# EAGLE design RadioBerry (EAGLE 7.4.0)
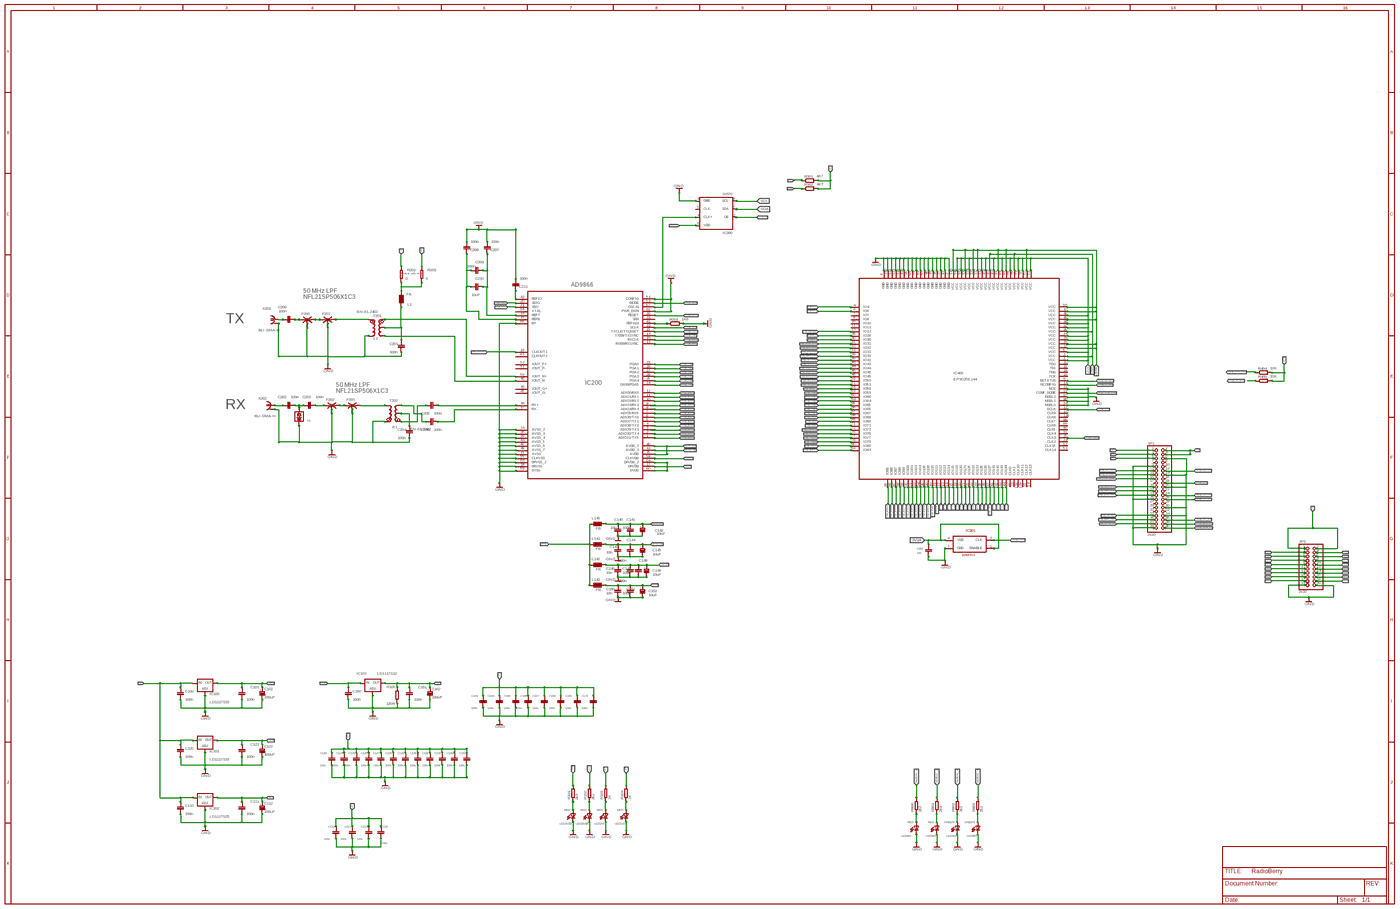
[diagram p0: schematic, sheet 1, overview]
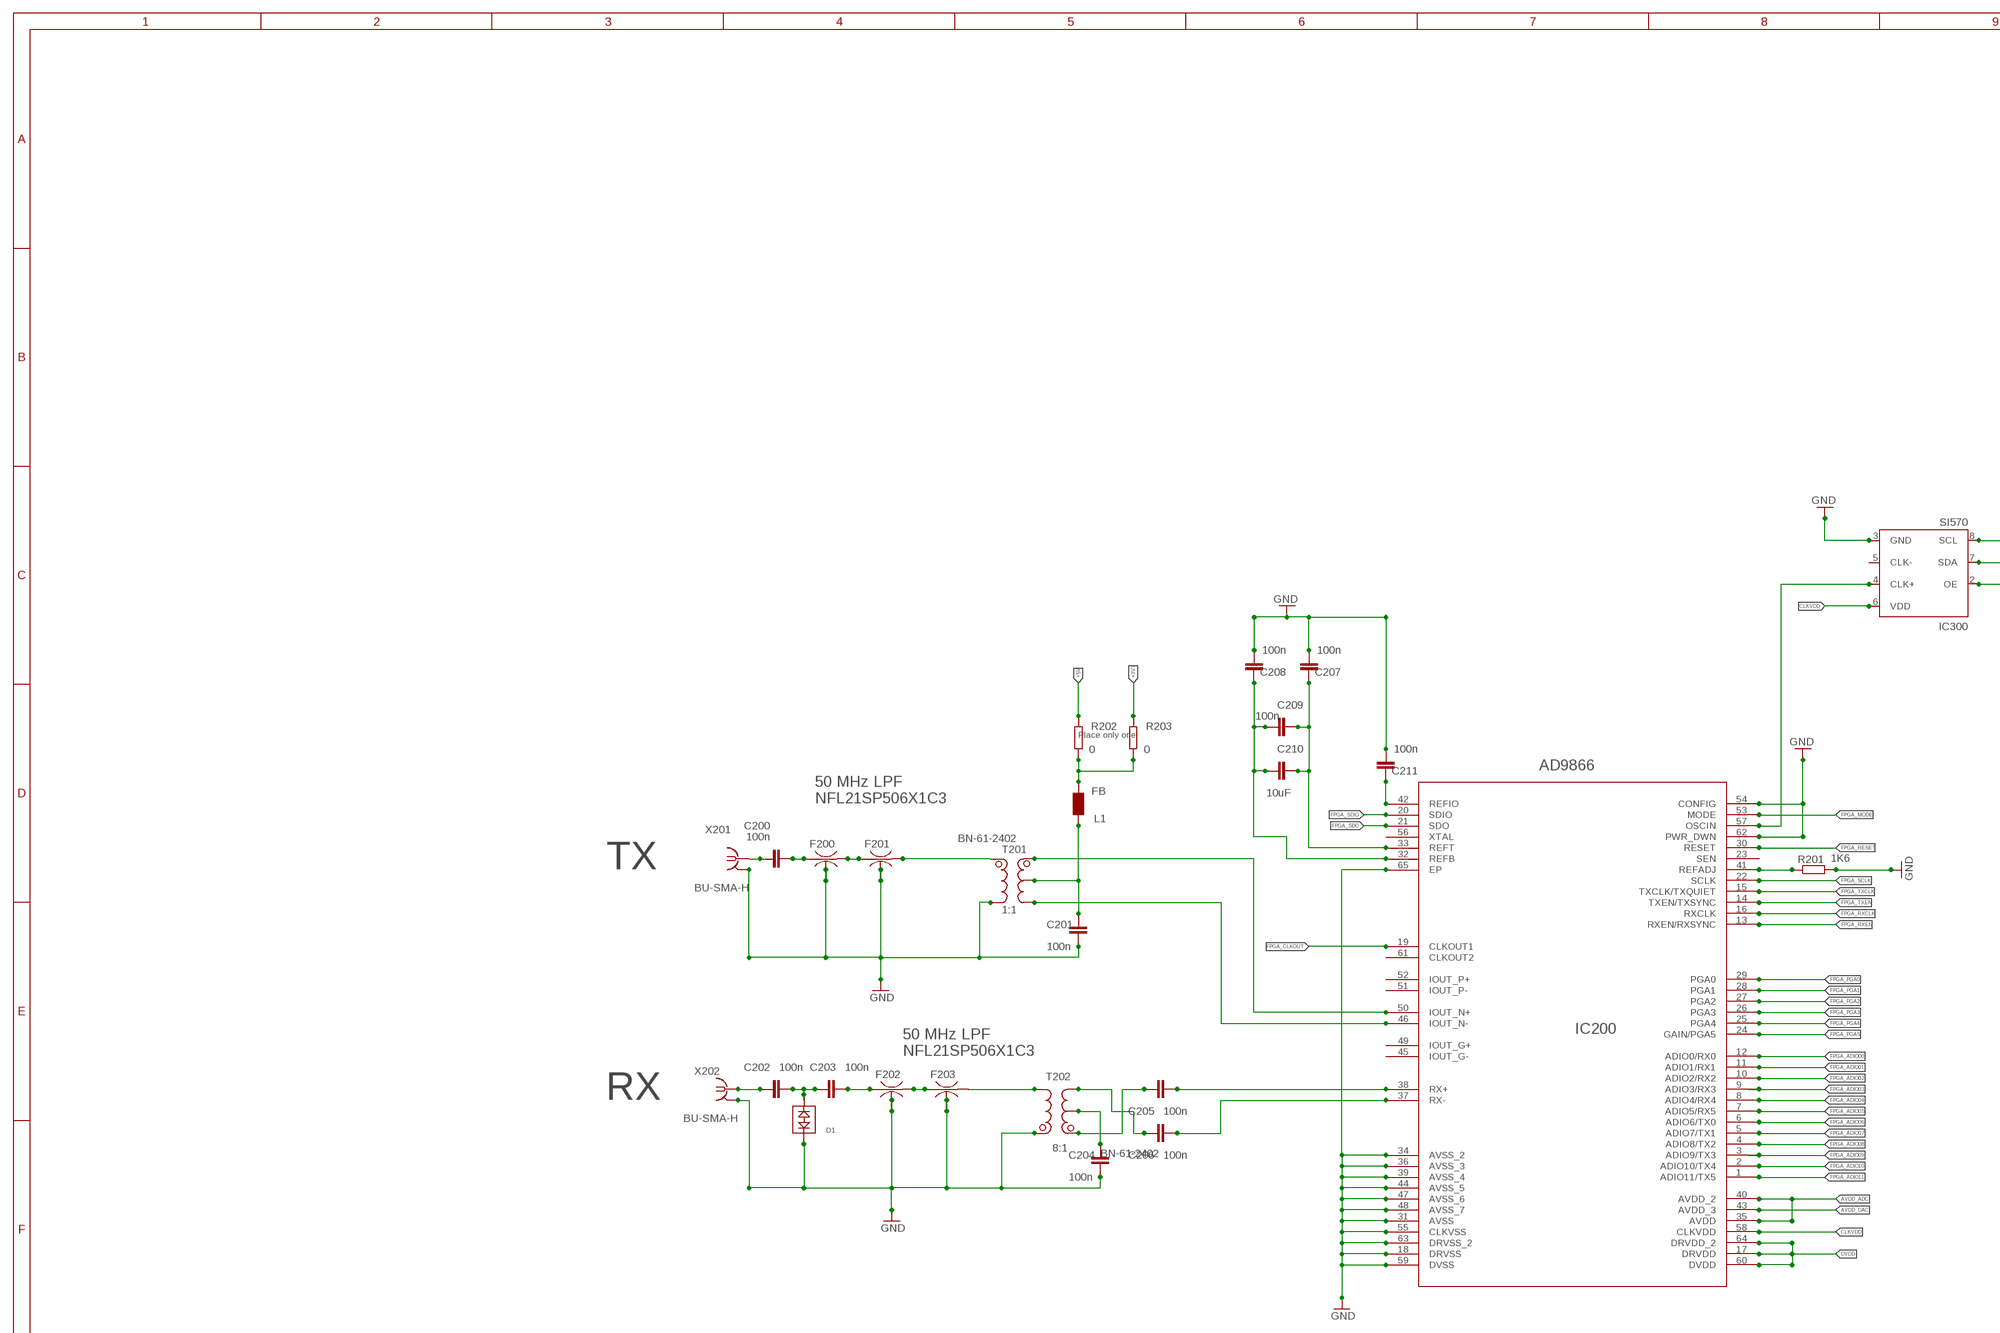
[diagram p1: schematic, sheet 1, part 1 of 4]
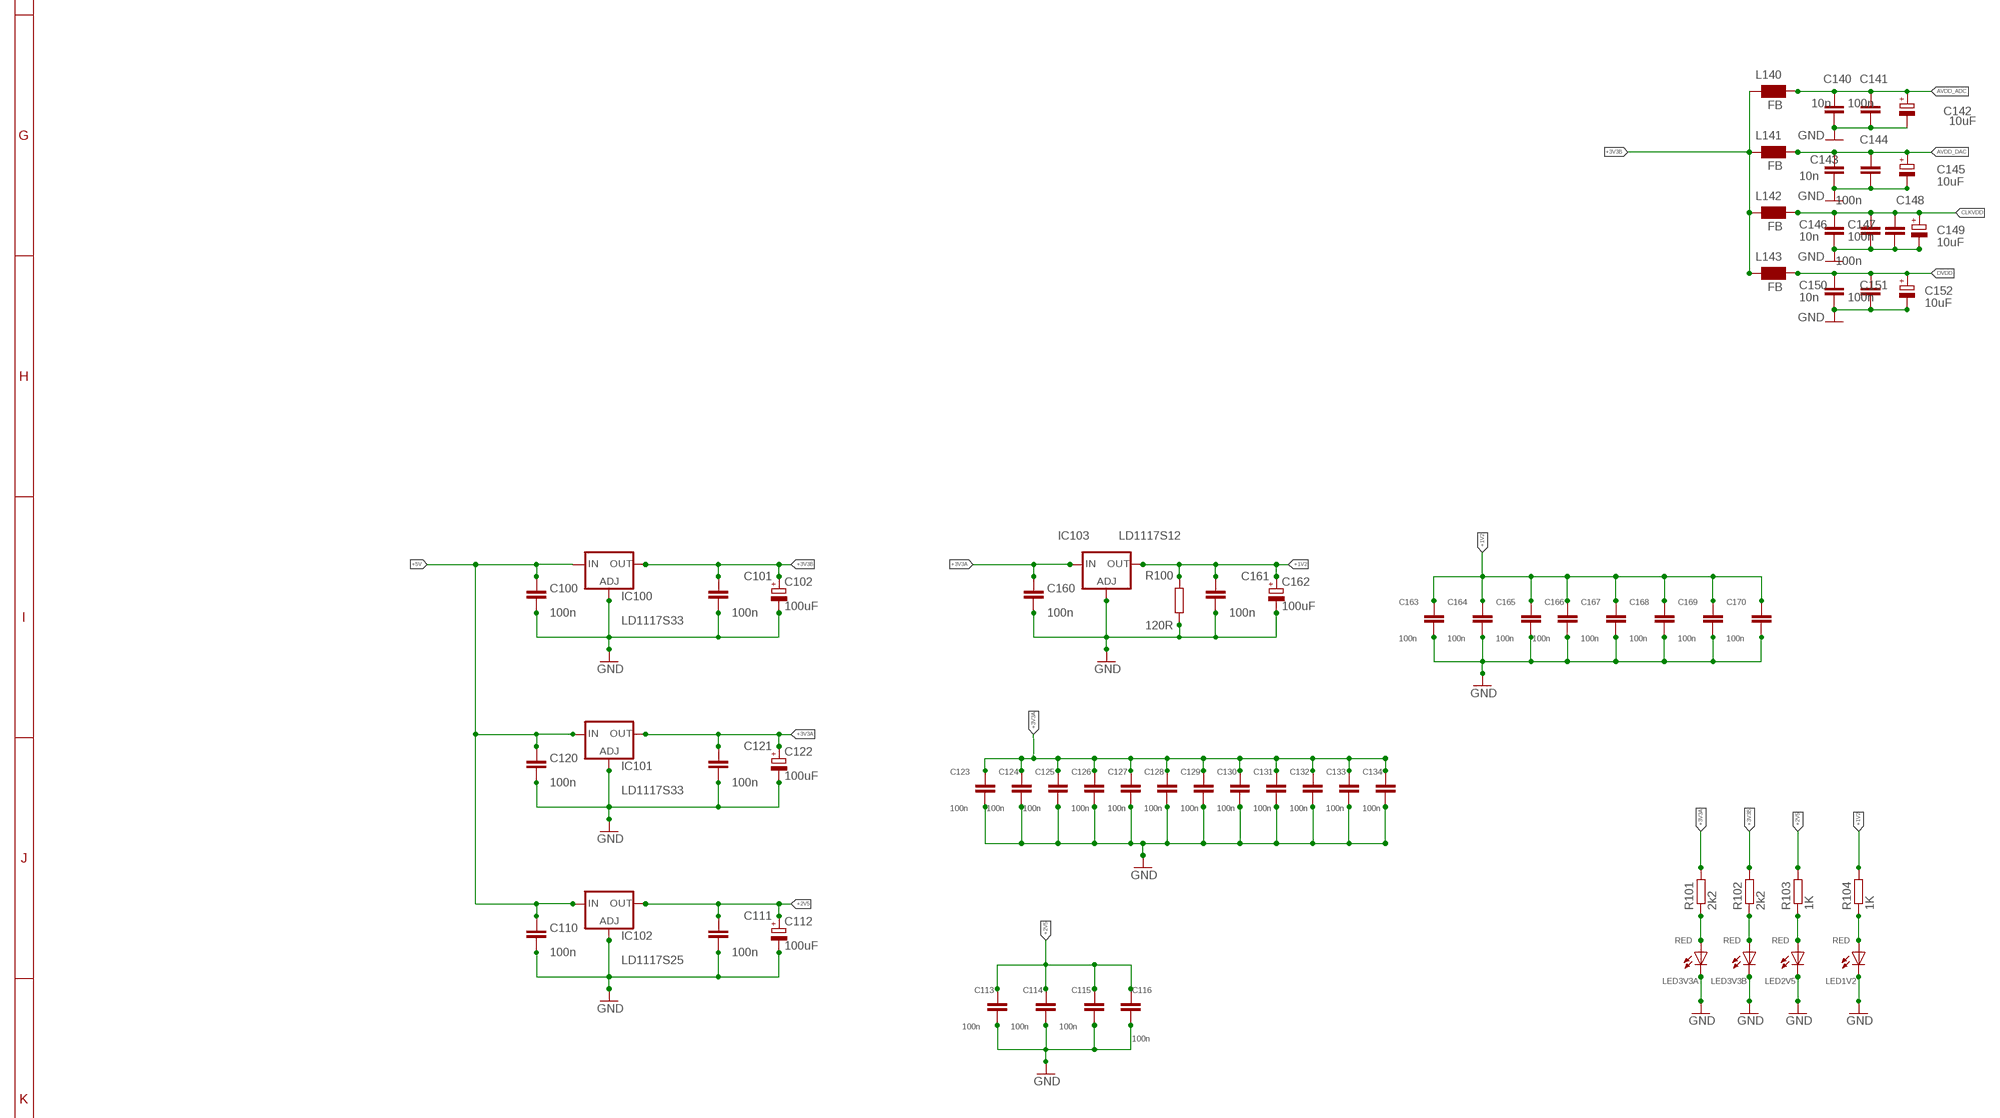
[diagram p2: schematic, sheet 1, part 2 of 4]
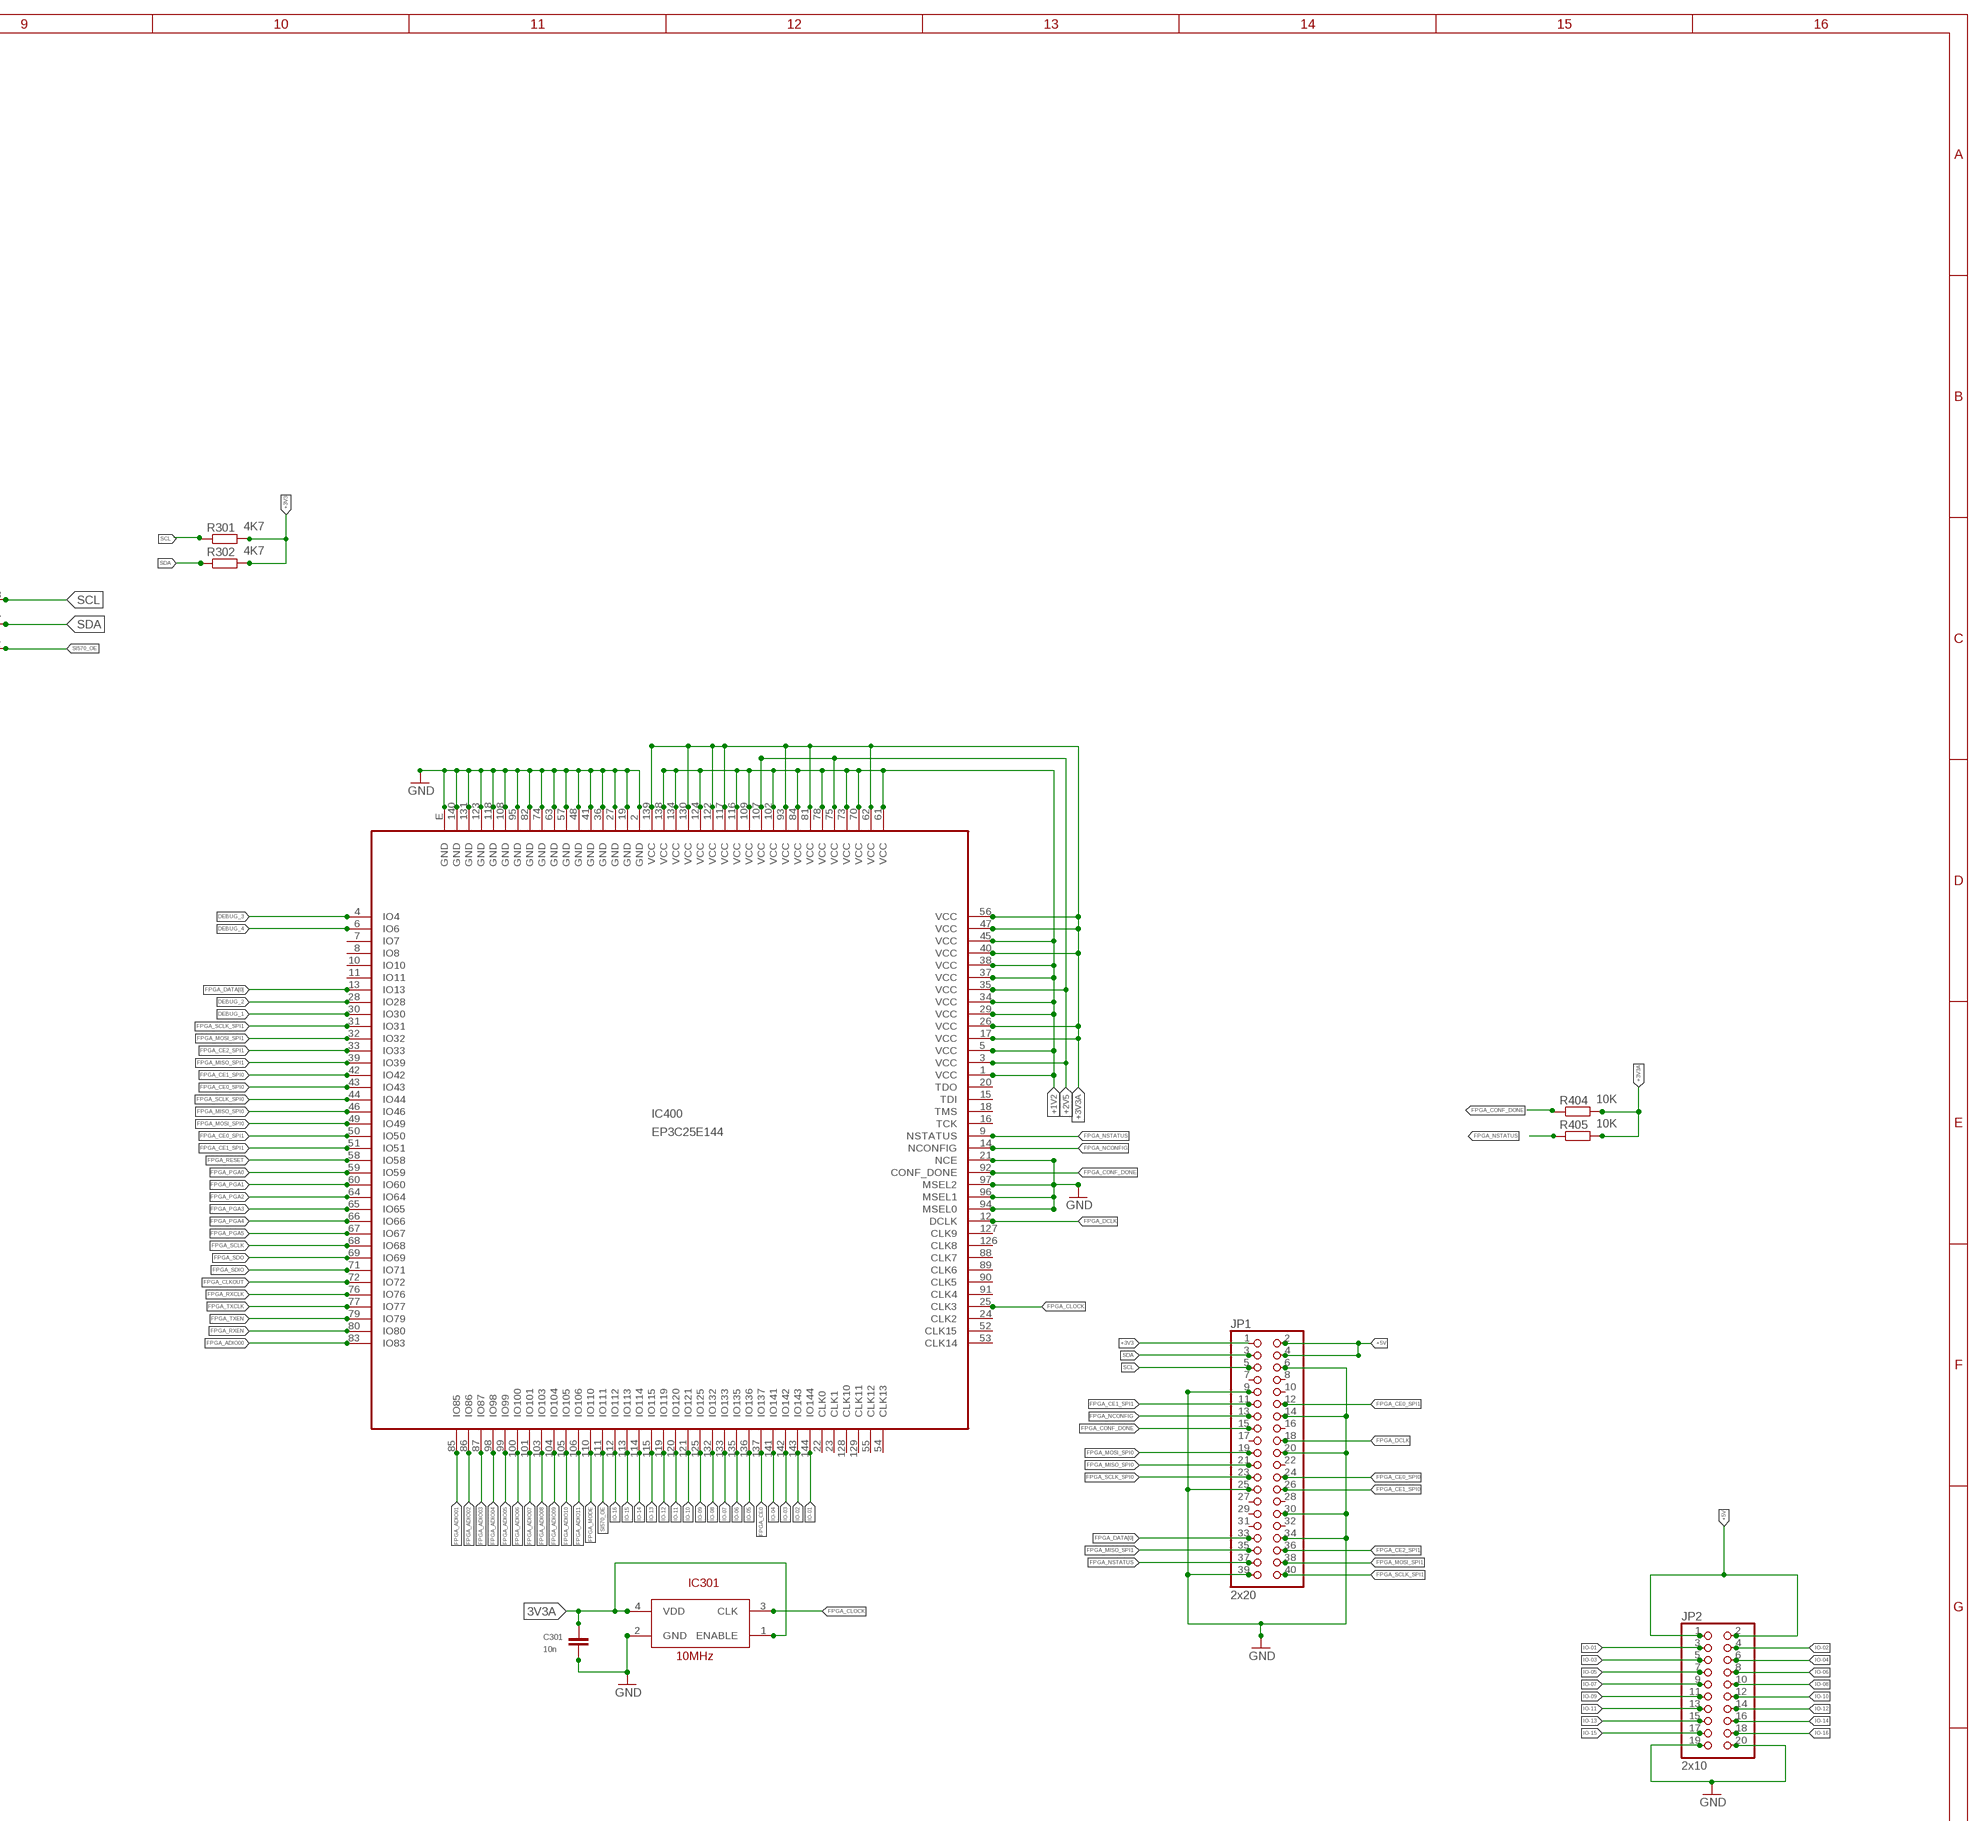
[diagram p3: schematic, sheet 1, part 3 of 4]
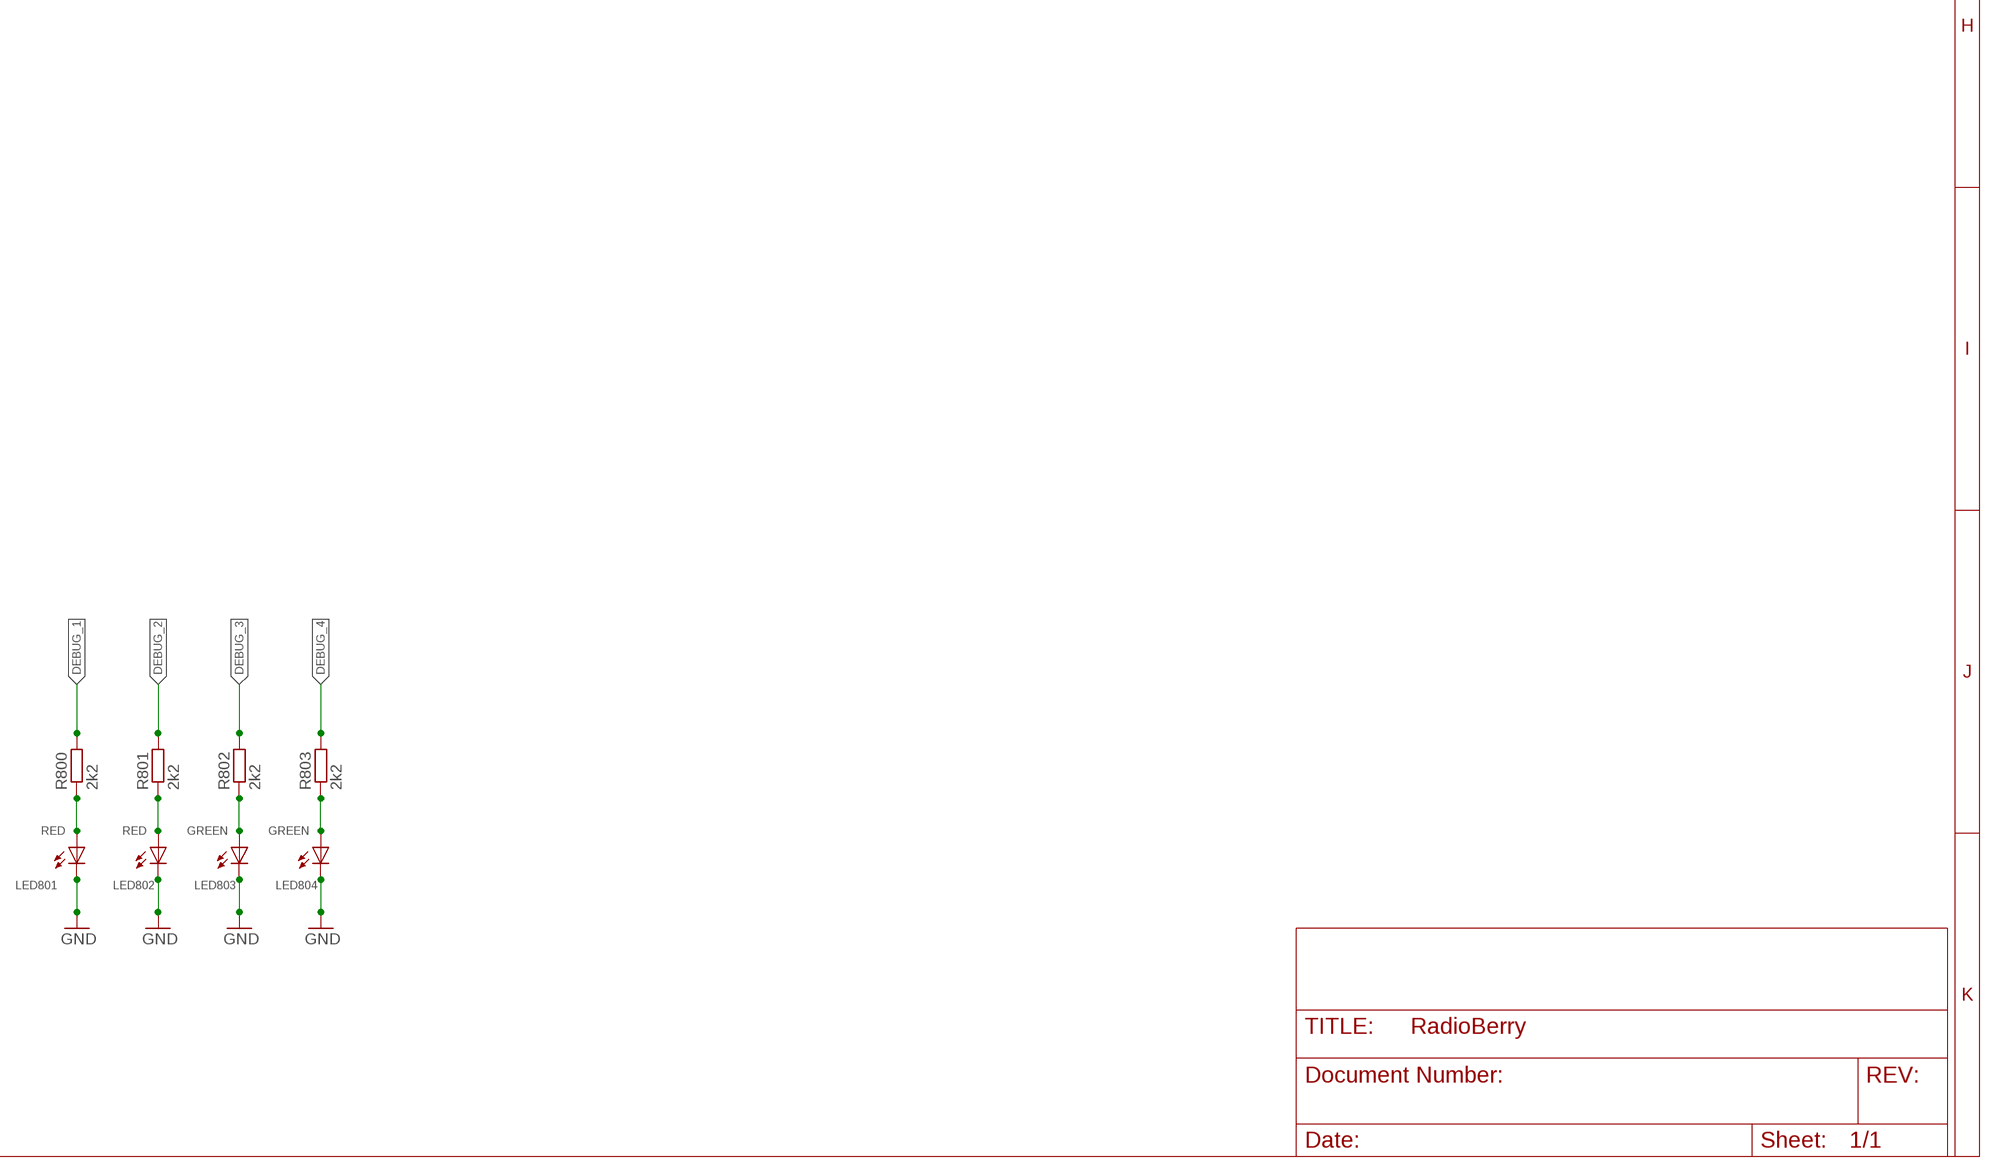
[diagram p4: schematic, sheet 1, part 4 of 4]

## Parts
C100  100n  C-EUC0603  [C0603]
C101  100n  C-EUC0603  [C0603]
C102  100uF  CPOL-EUSMCA  [SMC_A]
C110  100n  C-EUC0603  [C0603]
C111  100n  C-EUC0603  [C0603]
C112  100uF  CPOL-EUSMCA  [SMC_A]
C113  100n  C-EUC0603  [C0603]
C114  100n  C-EUC0603  [C0603]
C115  100n  C-EUC0603  [C0603]
C116  100n  C-EUC0603  [C0603]
C120  100n  C-EUC0603  [C0603]
C121  100n  C-EUC0603  [C0603]
C122  100uF  CPOL-EUSMCA  [SMC_A]
C123  100n  C-EUC0603  [C0603]
C124  100n  C-EUC0603  [C0603]
C125  100n  C-EUC0603  [C0603]
C126  100n  C-EUC0603  [C0603]
C127  100n  C-EUC0603  [C0603]
C128  100n  C-EUC0603  [C0603]
C129  100n  C-EUC0603  [C0603]
C130  100n  C-EUC0603  [C0603]
C131  100n  C-EUC0603  [C0603]
C132  100n  C-EUC0603  [C0603]
C133  100n  C-EUC0603  [C0603]
C134  100n  C-EUC0603  [C0603]
C140  10n  C-EUC0603  [C0603]
C141  100n  C-EUC0603  [C0603]
C142  10uF  CPOL-EUSMCA  [SMC_A]
C143  10n  C-EUC0603  [C0603]
C144  100n  C-EUC0603  [C0603]
C145  10uF  CPOL-EUSMCA  [SMC_A]
C146  10n  C-EUC0603  [C0603]
C147  100n  C-EUC0603  [C0603]
C148  100n  C-EUC0603  [C0603]
C149  10uF  CPOL-EUSMCA  [SMC_A]
C150  10n  C-EUC0603  [C0603]
C151  100n  C-EUC0603  [C0603]
C152  10uF  CPOL-EUSMCA  [SMC_A]
C160  100n  C-EUC0603  [C0603]
C161  100n  C-EUC0603  [C0603]
C162  100uF  CPOL-EUSMCA  [SMC_A]
C163  100n  C-EUC0603  [C0603]
C164  100n  C-EUC0603  [C0603]
C165  100n  C-EUC0603  [C0603]
C166  100n  C-EUC0603  [C0603]
C167  100n  C-EUC0603  [C0603]
C168  100n  C-EUC0603  [C0603]
C169  100n  C-EUC0603  [C0603]
C170  100n  C-EUC0603  [C0603]
C200  100n  C-EUC0603  [C0603]
C201  100n  C-EUC0603  [C0603]
C202  100n  C-EUC0603  [C0603]
C203  100n  C-EUC0603  [C0603]
C204  100n  C-EUC0603  [C0603]
C205  100n  C-EUC0603  [C0603]
C206  100n  C-EUC0603  [C0603]
C207  100n  C-EUC0603  [C0603]
C208  100n  C-EUC0603  [C0603]
C209  100n  C-EUC0603  [C0603]
C210  10uF  C-EUC1206  [C1206]
C211  100n  C-EUC0603  [C0603]
C301  10n  C-EUC0603  [C0603]
D1  GBLC03C  [SOD-323]
F200  NFM21C  [NFM21C]
F201  NFM21C  [NFM21C]
F202  NFM21C  [NFM21C]
F203  NFM21C  [NFM21C]
IC100  LD1117S33  LD117AS33TR  [SOT223]
IC101  LD1117S33  LD117AS33TR  [SOT223]
IC102  LD1117S25  LD117AS33TR  [SOT223]
IC103  LD1117S12  LD117AS12TR  [SOT223]
IC200  AD9866  [CP_64_3]
IC300  SI570  [8-PIN]
IC301  10MHz  CLOCK  [MODEL625]
IC400  EP3C25E144  [EQFP144]
JP1  2x20  PINHD-2X20  [2X20]
JP2  2x10  PINHD-2X10  [2X10]
L1  FB  WE-CBF_0805  [0805]
L140  FB  WE-CBF_0805  [0805]
L141  FB  WE-CBF_0805  [0805]
L142  FB  WE-CBF_0805  [0805]
L143  FB  WE-CBF_0805  [0805]
LED1V2  RED  LEDCHIP-LED0805  [CHIP-LED0805]
LED2V5  RED  LEDCHIP-LED0805  [CHIP-LED0805]
LED3V3A  RED  LEDCHIP-LED0805  [CHIP-LED0805]
LED3V3B  RED  LEDCHIP-LED0805  [CHIP-LED0805]
LED801  RED  LEDCHIP-LED0805  [CHIP-LED0805]
LED802  RED  LEDCHIP-LED0805  [CHIP-LED0805]
LED803  GREEN  LEDCHIP-LED0805  [CHIP-LED0805]
LED804  GREEN  LEDCHIP-LED0805  [CHIP-LED0805]
R100  120R  R-EU_R0805  [R0805]
R101  2k2  R-EU_R0805  [R0805]
R102  2k2  R-EU_R0805  [R0805]
R103  1K  R-EU_R0805  [R0805]
R104  1K  R-EU_R0805  [R0805]
R201  1K6  R-EU_R0805  [R0805]
R202  0  R-EU_R0805  [R0805]
R203  0  R-EU_R0805  [R0805]
R301  4K7  R-EU_R0805  [R0805]
R302  4K7  R-EU_R0805  [R0805]
R404  10K  R-EU_R0805  [R0805]
R405  10K  R-EU_R0805  [R0805]
R800  2k2  R-EU_R0805  [R0805]
R801  2k2  R-EU_R0805  [R0805]
R802  2k2  R-EU_R0805  [R0805]
R803  2k2  R-EU_R0805  [R0805]
T201  BN-61-2402  T1-1TDIL  [DIL06]
T202  BN-61-2402  T1-1TDIL  [DIL06]
X201  BU-SMA-H  [BU-SMA-H]
X202  BU-SMA-H  [BU-SMA-H]

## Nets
3V3A: C301.2 IC301.1(ENABLE) IC301.4(VDD)
+1V2: C161.2 C162.+ C163.2 C164.2 C165.2 C166.2 C167.2 C168.2 C169.2 C170.2 IC103.4(OUT) IC400.1(VCC) IC400.5(VCC) IC400.29(VCC) IC400.34(VCC) IC400.37(VCC) IC400.38(VCC) IC400.45(VCC) IC400.61(VCC) IC400.70(VCC) IC400.73(VCC) IC400.78(VCC) IC400.84(VCC) IC400.102(VCC) IC400.109(VCC) IC400.116(VCC) IC400.124(VCC) IC400.134(VCC) IC400.138(VCC) R100.2 R104.2
+2V5: C111.2 C112.+ C113.2 C114.2 C115.2 C116.2 IC102.4(OUT) IC400.3(VCC) IC400.35(VCC) IC400.75(VCC) IC400.107(VCC) R103.2
+3V3: JP1.1 R203.2 R301.2 R302.2
+3V3A: C121.2 C122.+ C123.2 C124.2 C125.2 C126.2 C127.2 C128.2 C129.2 C130.2 C131.2 C132.2 C133.2 C134.2 C160.2 IC101.4(OUT) IC103.3(IN) IC400.17(VCC) IC400.26(VCC) IC400.40(VCC) IC400.47(VCC) IC400.56(VCC) IC400.62(VCC) IC400.81(VCC) IC400.93(VCC) IC400.117(VCC) IC400.122(VCC) IC400.130(VCC) IC400.139(VCC) R101.2 R404.2 R405.2
+3V3B: C101.2 C102.+ IC100.4(OUT) L140.1 L141.1 L142.1 L143.1 R102.2
+5V: C100.2 C110.2 C120.2 IC100.3(IN) IC101.3(IN) IC102.3(IN) JP1.2 JP1.4 JP2.1 JP2.2 R202.2
AVDD_ADC: C140.2 C141.2 C142.+ IC200.35(AVDD) IC200.40(AVDD_2) L140.2
AVDD_DAC: C143.2 C144.2 C145.+ IC200.43(AVDD_3) L141.2
CLK: IC200.57(OSCIN) IC300.4(CLK+)
CLKVDD: C146.2 C147.2 C148.2 C149.+ IC200.58(CLKVDD) IC300.6(VDD) L142.2
DEBUG_1: IC400.30(IO30) R800.2
DEBUG_2: IC400.28(IO28) R801.2
DEBUG_3: IC400.4(IO4) R802.2
DEBUG_4: IC400.6(IO6) R803.2
DVDD: C150.2 C151.2 C152.+ IC200.17(DRVDD) IC200.60(DVDD) IC200.64(DRVDD_2) L143.2
FPGA_ADIO00: IC200.12(ADIO0/RX0) IC400.83(IO83)
FPGA_ADIO01: IC200.11(ADIO1/RX1) IC400.85(IO85)
FPGA_ADIO02: IC200.10(ADIO2/RX2) IC400.86(IO86)
FPGA_ADIO03: IC200.9(ADIO3/RX3) IC400.87(IO87)
FPGA_ADIO04: IC200.8(ADIO4/RX4) IC400.98(IO98)
FPGA_ADIO05: IC200.7(ADIO5/RX5) IC400.99(IO99)
FPGA_ADIO06: IC200.6(ADIO6/TX0) IC400.100(IO100)
FPGA_ADIO07: IC200.5(ADIO7/TX1) IC400.101(IO101)
FPGA_ADIO08: IC200.4(ADIO8/TX2) IC400.103(IO103)
FPGA_ADIO09: IC200.3(ADIO9/TX3) IC400.104(IO104)
FPGA_ADIO10: IC200.2(ADIO10/TX4) IC400.105(IO105)
FPGA_ADIO11: IC200.1(ADIO11/TX5) IC400.106(IO106)
FPGA_CE0: IC400.137(IO137)
FPGA_CE0_SPI0: IC400.43(IO43) JP1.24
FPGA_CE0_SPI1: IC400.50(IO50) JP1.12
FPGA_CE1_SPI0: IC400.42(IO42) JP1.26
FPGA_CE1_SPI1: IC400.51(IO51) JP1.11
FPGA_CE2_SPI1: IC400.33(IO33) JP1.36
FPGA_CLKOUT: IC200.19(CLKOUT1) IC400.72(IO72)
FPGA_CLOCK: IC301.3(CLK) IC400.25(CLK3)
FPGA_CONF_DONE: IC400.92(CONF_DONE) JP1.15 R404.1
FPGA_DATA[0]: IC400.13(IO13) JP1.33
FPGA_DCLK: IC400.12(DCLK) JP1.18
FPGA_MISO_SPI0: IC400.46(IO46) JP1.21
FPGA_MISO_SPI1: IC400.39(IO39) JP1.35
FPGA_MODE: IC200.53(MODE) IC400.110(IO110)
FPGA_MOSI_SPI0: IC400.49(IO49) JP1.19
FPGA_MOSI_SPI1: IC400.32(IO32) JP1.38
FPGA_NCONFIG: IC400.14(NCONFIG) JP1.13
FPGA_NSTATUS: IC400.9(NSTATUS) JP1.37 R405.1
FPGA_PGA0: IC200.29(PGA0) IC400.59(IO59)
FPGA_PGA1: IC200.28(PGA1) IC400.60(IO60)
FPGA_PGA2: IC200.27(PGA2) IC400.64(IO64)
FPGA_PGA3: IC200.26(PGA3) IC400.65(IO65)
FPGA_PGA4: IC200.25(PGA4) IC400.66(IO66)
FPGA_PGA5: IC200.24(GAIN/PGA5) IC400.67(IO67)
FPGA_RESET: IC200.30(RESET) IC400.58(IO58)
FPGA_RXCLK: IC200.16(RXCLK) IC400.76(IO76)
FPGA_RXEN: IC200.13(RXEN/RXSYNC) IC400.80(IO80)
FPGA_SCLK: IC200.22(SCLK) IC400.68(IO68)
FPGA_SCLK_SPI0: IC400.44(IO44) JP1.23
FPGA_SCLK_SPI1: IC400.31(IO31) JP1.40
FPGA_SDIO: IC200.20(SDIO) IC400.71(IO71)
FPGA_SDO: IC200.21(SDO) IC400.69(IO69)
FPGA_TXCLK: IC200.15(TXCLK/TXQUIET) IC400.77(IO77)
FPGA_TXEN: IC200.14(TXEN/TXSYNC) IC400.79(IO79)
GND: C100.1 C101.1 C102.- C110.1 C111.1 C112.- C113.1 C114.1 C115.1 C116.1 C120.1 C121.1 C122.- C123.1 C124.1 C125.1 C126.1 C127.1 C128.1 C129.1 C130.1 C131.1 C132.1 C133.1 C134.1 C140.1 C141.1 C142.- C143.1 C144.1 C145.- C146.1 C147.1 C148.1 C149.- C150.1 C151.1 C152.- C160.1 C161.1 C162.- C163.1 C164.1 C165.1 C166.1 C167.1 C168.1 C169.1 C170.1 C201.1 C204.1 C207.1 C208.1 C211.1 C301.1 D1.B F200.2@1 F200.2@2 F201.2@1 F201.2@2 F202.2@1 F202.2@2 F203.2@1 F203.2@2 IC100.1(ADJ) IC101.1(ADJ) IC102.1(ADJ) IC103.1(ADJ) IC200.18(DRVSS) IC200.31(AVSS) IC200.34(AVSS_2) IC200.36(AVSS_3) IC200.39(AVSS_4) IC200.44(AVSS_5) IC200.47(AVSS_6) IC200.48(AVSS_7) IC200.54(CONFIG) IC200.55(CLKVSS) IC200.59(DVSS) IC200.62(PWR_DWN) IC200.63(DRVSS_2) IC200.65(EP) IC300.3(GND) IC301.2(GND) IC400.2(GND) IC400.19(GND) IC400.21(NCE) IC400.27(GND) IC400.36(GND) IC400.41(GND) IC400.48(GND) IC400.57(GND) IC400.63(GND) IC400.74(GND) IC400.82(GND) IC400.94(MSEL0) IC400.95(GND) IC400.96(MSEL1) IC400.97(MSEL2) IC400.108(GND) IC400.118(GND) IC400.123(GND) IC400.131(GND) IC400.140(GND) IC400.E(GND) JP1.6 JP1.9 JP1.14 JP1.20 JP1.25 JP1.30 JP1.34 JP1.39 JP2.19 JP2.20 LED1V2.C LED2V5.C LED3V3A.C LED3V3B.C LED801.C LED802.C LED803.C LED804.C R100.1 R201.2 T201.1(P2) T202.3(P1) X201.2 X201.3 X201.4 X201.5 X202.2 X202.3 X202.4 X202.5
IO-01: IC400.144(IO144) JP2.3
IO-02: IC400.143(IO143) JP2.4
IO-03: IC400.142(IO142) JP2.5
IO-04: IC400.141(IO141) JP2.6
IO-05: IC400.136(IO136) JP2.7
IO-06: IC400.135(IO135) JP2.8
IO-07: IC400.133(IO133) JP2.9
IO-08: IC400.132(IO132) JP2.10
IO-09: IC400.125(IO125) JP2.11
IO-10: IC400.121(IO121) JP2.12
IO-11: IC400.120(IO120) JP2.13
IO-12: IC400.119(IO119) JP2.14
IO-13: IC400.115(IO115) JP2.15
IO-14: IC400.114(IO114) JP2.16
IO-15: IC400.113(IO113) JP2.17
IO-16: IC400.112(IO112) JP2.18
N$1: L1.2 R202.1 R203.1
N$2: F203.3 T202.1(P2)
N$3: C205.2 T202.4(S1)
N$4: C201.2 L1.1 T201.5(ST)
N$5: C202.1 C203.2 D1.A
N$6: IC200.50(IOUT_N+) T201.4(S1)
N$7: IC200.46(IOUT_N-) T201.6(S2)
N$8: C206.2 T202.6(S2)
N$10: LED3V3B.A R102.1
N$11: LED2V5.A R103.1
N$13: C206.1 IC200.37(RX-)
N$14: C204.2 T202.5(ST)
N$15: C205.1 IC200.38(RX+)
N$16: LED801.A R800.1
N$17: LED802.A R801.1
N$18: LED803.A R802.1
N$19: LED804.A R803.1
N$20: LED3V3A.A R101.1
N$23: LED1V2.A R104.1
N$25: F202.3 F203.1
N$28: C202.2 X202.1
N$29: C203.1 F202.1
N$30: C207.2 C209.2 C210.2 IC200.33(REFT)
N$32: C208.2 C209.1 C210.1 IC200.32(REFB)
N$33: C211.2 IC200.42(REFIO)
N$34: IC200.41(REFADJ) R201.1
N$69: C200.2 X201.1
N$71: C200.1 F200.1
N$72: F200.3 F201.1
N$73: F201.3 T201.3(P1)
SCL: IC300.8(SCL) JP1.5 R301.1
SDA: IC300.7(SDA) JP1.3 R302.1
SI570_OE: IC300.2(OE) IC400.111(IO111)
Unconnected: IC200.23(SEN) IC200.45(IOUT_G-) IC200.49(IOUT_G+) IC200.51(IOUT_P-) IC200.52(IOUT_P+) IC200.56(XTAL) IC200.61(CLKOUT2) IC300.5(CLK-) IC400.7(IO7) IC400.8(IO8) IC400.10(IO10) IC400.11(IO11) IC400.15(TDI) IC400.16(TCK) IC400.18(TMS) IC400.20(TDO) IC400.22(CLK0) IC400.23(CLK1) IC400.24(CLK2) IC400.52(CLK15) IC400.53(CLK14) IC400.54(CLK13) IC400.55(CLK12) IC400.88(CLK7) IC400.89(CLK6) IC400.90(CLK5) IC400.91(CLK4) IC400.126(CLK8) IC400.127(CLK9) IC400.128(CLK10) IC400.129(CLK11) JP1.7 JP1.8 JP1.10 JP1.16 JP1.17 JP1.22 JP1.27 JP1.28 JP1.29 JP1.31 JP1.32

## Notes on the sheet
- Configuration
- Place only one
- 50 MHz LPF
  NFL21SP506X1C3
- TX
- 1:1
- 50 MHz LPF
  NFL21SP506X1C3
- RX
- 8:1
- Power Supply
- [100]

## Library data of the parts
C100 C101 C110 C111 C113-C116 C120 C121 C123-C134 C140 C141 C143 C144 C146-C148 C150 C151 C160 C161 C163-C170 C200-C211 C301 = rcl:C-EU: CAPACITOR, European symbol
C102 C112 C122 C142 C145 C149 C152 C162 = rcl:CPOL-EU: POLARIZED CAPACITOR, European symbol
D1 = pa3gsb:GBLC03C
F200-F203 = murata-filter:NFM: EMIFIL(R) (Capacitor type) Single Circuit Type for Signal Lines Source: http://search.murata.co.jp/Ceramy/image/img/PDF/ENG/L0111S0109NFM3DC.pdf
IC100-IC103 = v-reg:LD117A?*: Low drop fixed and adjustable positive voltage regulators 1 A Source: http://www.st.com/stonline/products/literature/ds/7194/ld1117axx.pdf
IC200 = AD9866:AD9866
IC300 = silabs:SI570: ANY-RATE I2C PROGRAMMABLE XO/VCXO Source: si570.pdf; OC_FARNELL: unknown; OC_NEWARK: unknown
IC301 = AVS-Clock:CLOCK
IC400 = altera-cyclone-III:EP3C25E144: EP3C25E144 edit this description Auto generated by make-symbol-device-package-bsdl.ulp Rev. 20 Source: EP3C25E144.bsd http://www.altera.com/support/devices/bsdl/cyclone3/cyc3-index.jsp; MPN: EP3C25E144C8N; OC_FARNELL: 1453474; OC_NEWARK: 51R0605
JP1 = pinhead:PINHD-2X20: PIN HEADER
JP2 = pinhead:PINHD-2X10: PIN HEADER
L1 L140-L143 = wuerth-elektronik:WE-CBF: SMD EMI Suppression Ferrite Beads
LED1V2 LED2V5 LED3V3A LED3V3B LED801-LED804 = led:LED: LED
R100-R104 R201-R203 R301 R302 R404 R405 R800-R803 = rcl:R-EU_: RESISTOR, European symbol
T201 T202 = pa3gsb:T1-1T
X201 X202 = con-coax:BU-SMA-H: FEMALE SMA CONNECTOR; OC_FARNELL: unknown; OC_NEWARK: unknown

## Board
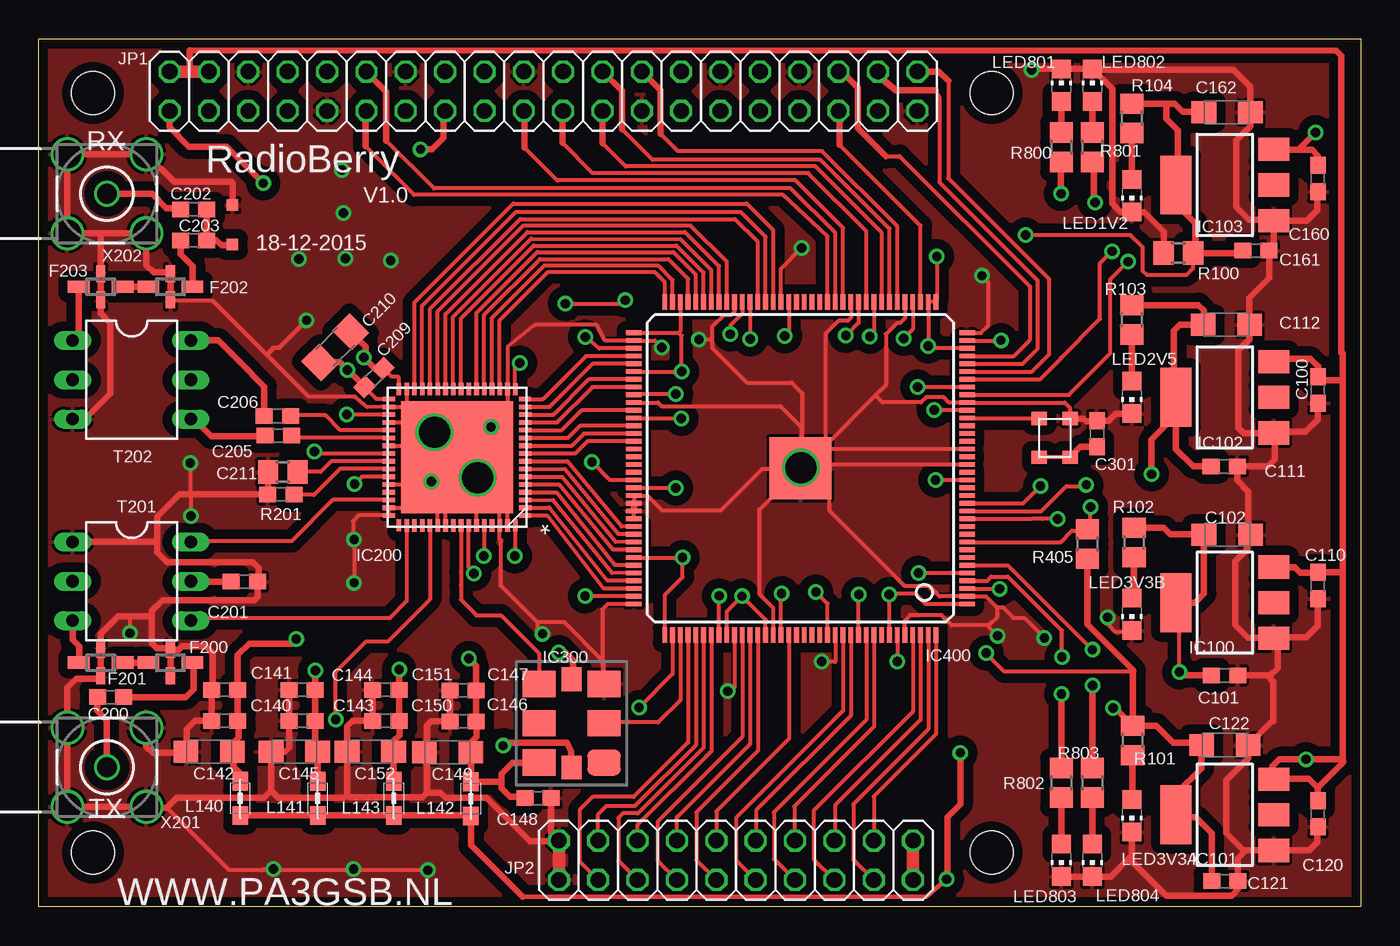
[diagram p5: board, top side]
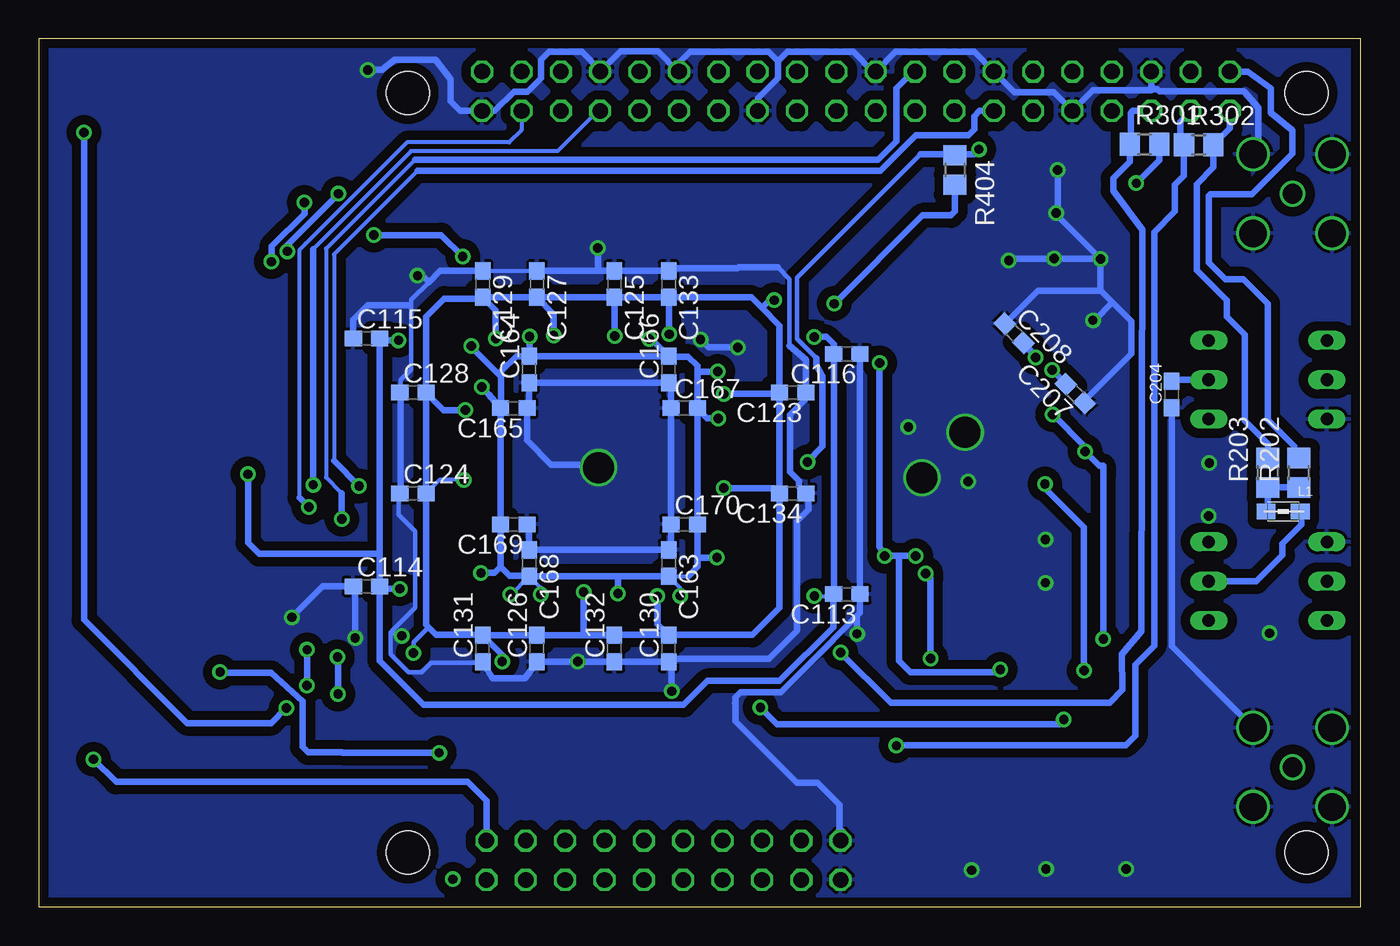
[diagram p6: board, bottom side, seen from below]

Size 85.32 x 56 mm. Coordinates in mm from the lower left corner, seen from the top.
Outline: 0,56 85.32,56 85.32,0 0,0 0,56
Copper layers (1*16): Top 0.018mm / dielectric 1.55mm / Bottom 0.018mm
Design rules "eC-PCB_proto-2-layer": minimum track width 0.15mm, minimum drill 0.25mm, track to track 0.15mm, track to pad 0.15mm, pad to pad 0.15mm, via to via 0.15mm, smd to smd 0.15mm, copper to edge 0.45mm, drill to drill 0.3mm, minimum pad ring 0.2mm, minimum via ring 0.2mm, stop-mask expansion 0.1mm, vias tented up to drill 0mil, thermal gap 0.2mm
Holes 2.75 mm at 3.5,52.5 61.5,52.5 3.5,3.5 61.5,3.5

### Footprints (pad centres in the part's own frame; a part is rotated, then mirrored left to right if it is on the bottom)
C0603 = smd 1.1 x 1: 1 -0.85,0; 2 0.85,0
SMC_A = smd 1.6 x 1.4: + -1.5,0; - 1.5,0
C1206 = smd 1.6 x 1.8: 1 -1.4,0; 2 1.4,0
SOD-323 = smd 0.762 x 0.762: A -1.27,0; B 1.27,0
NFM21C = smd 1.4 x 0.8: 1 -1.425,0; 3 1.425,0 | smd 0.6 x 1.1: 2@1 0,-0.85; 2@2 0,0.85
SOT223 = smd 1.5 x 2: 1 -2.3,-3.15; 2 0,-3.15; 3 2.3,-3.15 | smd 3.8 x 2: 4 0,3.15
CP_64_3 = smd 0.762 x 0.305: 1 -4.394,3.75; 16 -4.394,-3.75; 33 4.394,-3.75; 48 4.394,3.75 | smd 0.813 x 0.305: 2 -4.394,3.25; 3 -4.394,2.75; 4 -4.394,2.25; 5 -4.394,1.75; 6 -4.394,1.25; 7 -4.394,0.75; 8 -4.394,0.25; 9 -4.394,-0.25; 10 -4.394,-0.75; 11 -4.394,-1.25; 12 -4.394,-1.75; 13 -4.394,-2.25; 14 -4.394,-2.75; 15 -4.394,-3.25; 34 4.394,-3.25; 35 4.394,-2.75; 36 4.394,-2.25; 37 4.394,-1.75; 38 4.394,-1.25; 39 4.394,-0.75; 40 4.394,-0.25; 41 4.394,0.25; 42 4.394,0.75; 43 4.394,1.25; 44 4.394,1.75; 45 4.394,2.25; 46 4.394,2.75; 47 4.394,3.25 | smd 0.305 x 0.762: 17 -3.75,-4.394; 32 3.75,-4.394; 49 3.75,4.394; 64 -3.75,4.394 | smd 0.305 x 0.813: 18 -3.25,-4.394; 19 -2.75,-4.394; 20 -2.25,-4.394; 21 -1.75,-4.394; 22 -1.25,-4.394; 23 -0.75,-4.394; 24 -0.25,-4.394; 25 0.25,-4.394; 26 0.75,-4.394; 27 1.25,-4.394; 28 1.75,-4.394; 29 2.25,-4.394; 30 2.75,-4.394; 31 3.25,-4.394; 50 3.25,4.394; 51 2.75,4.394; 52 2.25,4.394; 53 1.75,4.394; 54 1.25,4.394; 55 0.75,4.394; 56 0.25,4.394; 57 -0.25,4.394; 58 -0.75,4.394; 59 -1.25,4.394; 60 -1.75,4.394; 61 -2.25,4.394; 62 -2.75,4.394; 63 -3.25,4.394 | smd 7.239 x 7.239: 65 0,0
8-PIN = smd 1.7 x 2.15: 1 -2.54,-2.1; 2 0,-2.1; 3 2.54,-2.1; 4 2.54,2.1; 5 0,2.1; 6 -2.54,2.1 | smd 1.545 x 1.3: 7 -2.853,0; 8 2.853,0
MODEL625 = smd 1 x 0.85: 1 -1,1.25; 2 -1,-1.25; 3 1,-1.25; 4 1,1.25
EQFP144 = smd 1 x 0.3: 1 -10.75,8.75; 2 -10.75,8.25; 3 -10.75,7.75; 4 -10.75,7.25; 5 -10.75,6.75; 6 -10.75,6.25; 7 -10.75,5.75; 8 -10.75,5.25; 9 -10.75,4.75; 10 -10.75,4.25; 11 -10.75,3.75; 12 -10.75,3.25; 13 -10.75,2.75; 14 -10.75,2.25; 15 -10.75,1.75; 16 -10.75,1.25; 17 -10.75,0.75; 18 -10.75,0.25; 19 -10.75,-0.25; 20 -10.75,-0.75; 21 -10.75,-1.25; 22 -10.75,-1.75; 23 -10.75,-2.25; 24 -10.75,-2.75; 25 -10.75,-3.25; 26 -10.75,-3.75; 27 -10.75,-4.25; 28 -10.75,-4.75; 29 -10.75,-5.25; 30 -10.75,-5.75; 31 -10.75,-6.25; 32 -10.75,-6.75; 33 -10.75,-7.25; 34 -10.75,-7.75; 35 -10.75,-8.25; 36 -10.75,-8.75; 73 10.75,-8.75; 74 10.75,-8.25; 75 10.75,-7.75; 76 10.75,-7.25; 77 10.75,-6.75; 78 10.75,-6.25; 79 10.75,-5.75; 80 10.75,-5.25; 81 10.75,-4.75; 82 10.75,-4.25; 83 10.75,-3.75; 84 10.75,-3.25; 85 10.75,-2.75; 86 10.75,-2.25; 87 10.75,-1.75; 88 10.75,-1.25; 89 10.75,-0.75; 90 10.75,-0.25; 91 10.75,0.25; 92 10.75,0.75; 93 10.75,1.25; 94 10.75,1.75; 95 10.75,2.25; 96 10.75,2.75; 97 10.75,3.25; 98 10.75,3.75; 99 10.75,4.25; 100 10.75,4.75; 101 10.75,5.25; 102 10.75,5.75; 103 10.75,6.25; 104 10.75,6.75; 105 10.75,7.25; 106 10.75,7.75; 107 10.75,8.25; 108 10.75,8.75 | smd 0.3 x 1: 37 -8.75,-10.75; 38 -8.25,-10.75; 39 -7.75,-10.75; 40 -7.25,-10.75; 41 -6.75,-10.75; 42 -6.25,-10.75; 43 -5.75,-10.75; 44 -5.25,-10.75; 45 -4.75,-10.75; 46 -4.25,-10.75; 47 -3.75,-10.75; 48 -3.25,-10.75; 49 -2.75,-10.75; 50 -2.25,-10.75; 51 -1.75,-10.75; 52 -1.25,-10.75; 53 -0.75,-10.75; 54 -0.25,-10.75; 55 0.25,-10.75; 56 0.75,-10.75; 57 1.25,-10.75; 58 1.75,-10.75; 59 2.25,-10.75; 60 2.75,-10.75; 61 3.25,-10.75; 62 3.75,-10.75; 63 4.25,-10.75; 64 4.75,-10.75; 65 5.25,-10.75; 66 5.75,-10.75; 67 6.25,-10.75; 68 6.75,-10.75; 69 7.25,-10.75; 70 7.75,-10.75; 71 8.25,-10.75; 72 8.75,-10.75; 109 8.75,10.75; 110 8.25,10.75; 111 7.75,10.75; 112 7.25,10.75; 113 6.75,10.75; 114 6.25,10.75; 115 5.75,10.75; 116 5.25,10.75; 117 4.75,10.75; 118 4.25,10.75; 119 3.75,10.75; 120 3.25,10.75; 121 2.75,10.75; 122 2.25,10.75; 123 1.75,10.75; 124 1.25,10.75; 125 0.75,10.75; 126 0.25,10.75; 127 -0.25,10.75; 128 -0.75,10.75; 129 -1.25,10.75; 130 -1.75,10.75; 131 -2.25,10.75; 132 -2.75,10.75; 133 -3.25,10.75; 134 -3.75,10.75; 135 -4.25,10.75; 136 -4.75,10.75; 137 -5.25,10.75; 138 -5.75,10.75; 139 -6.25,10.75; 140 -6.75,10.75; 141 -7.25,10.75; 142 -7.75,10.75; 143 -8.25,10.75; 144 -8.75,10.75 | smd 4 x 4: E 0,0
2X20 = drill 1.016 octagon: 1 -24.13,-1.27; 2 -24.13,1.27; 3 -21.59,-1.27; 4 -21.59,1.27; 5 -19.05,-1.27; 6 -19.05,1.27; 7 -16.51,-1.27; 8 -16.51,1.27; 9 -13.97,-1.27; 10 -13.97,1.27; 11 -11.43,-1.27; 12 -11.43,1.27; 13 -8.89,-1.27; 14 -8.89,1.27; 15 -6.35,-1.27; 16 -6.35,1.27; 17 -3.81,-1.27; 18 -3.81,1.27; 19 -1.27,-1.27; 20 -1.27,1.27; 21 1.27,-1.27; 22 1.27,1.27; 23 3.81,-1.27; 24 3.81,1.27; 25 6.35,-1.27; 26 6.35,1.27; 27 8.89,-1.27; 28 8.89,1.27; 29 11.43,-1.27; 30 11.43,1.27; 31 13.97,-1.27; 32 13.97,1.27; 33 16.51,-1.27; 34 16.51,1.27; 35 19.05,-1.27; 36 19.05,1.27; 37 21.59,-1.27; 38 21.59,1.27; 39 24.13,-1.27; 40 24.13,1.27
2X10 = drill 1.016 octagon: 1 -11.43,-1.27; 2 -11.43,1.27; 3 -8.89,-1.27; 4 -8.89,1.27; 5 -6.35,-1.27; 6 -6.35,1.27; 7 -3.81,-1.27; 8 -3.81,1.27; 9 -1.27,-1.27; 10 -1.27,1.27; 11 1.27,-1.27; 12 1.27,1.27; 13 3.81,-1.27; 14 3.81,1.27; 15 6.35,-1.27; 16 6.35,1.27; 17 8.89,-1.27; 18 8.89,1.27; 19 11.43,-1.27; 20 11.43,1.27
0805 = smd 1.2 x 1: 1 -1.1,0; 2 1.1,0
CHIP-LED0805 = smd 1.2 x 1.2: A 0,-1.05; C 0,1.05
R0805 = smd 1.3 x 1.5: 1 -0.95,0; 2 0.95,0
DIL06 = drill 0.813 long: 1 -2.54,-3.81; 2 0,-3.81; 3 2.54,-3.81; 4 2.54,3.81; 5 0,3.81; 6 -2.54,3.81
BU-SMA-H = drill 1.27: 1 0,0 | drill 1.778: 2 -2.55,2.55; 3 2.55,2.55; 4 2.55,-2.55; 5 -2.55,-2.55

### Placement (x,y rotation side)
C100  82.55,33.33 90 top
C101  76.53,14.93 180 top
C102  76.7,24 0 top
C110  82.55,20.72 90 top
C111  76.51,28.41 180 top
C112  76.64,37.55 0 top
C113  33.16,20.17 180 bottom
C114  64.16,20.67 0 bottom
C115  64.16,36.67 0 bottom
C116  33.16,35.67 180 bottom
C120  82.55,6 90 top
C121  76.55,1.66 180 top
C122  76.55,10.43 0 top
C123  36.66,33.17 180 bottom
C124  61.16,26.67 0 bottom
C125  48.16,40.17 270 bottom
C126  53.16,16.67 90 bottom
C127  53.16,40.17 270 bottom
C128  61.16,33.17 0 bottom
C129  56.66,40.17 270 bottom
C130  44.66,16.67 90 bottom
C131  56.66,16.67 90 bottom
C132  48.16,16.67 90 bottom
C133  44.66,40.17 270 bottom
C134  36.66,26.67 180 bottom
C140  12,12 0 top
C141  12,14 0 top
C142  11,10 180 top
C143  17,12 0 top
C144  17,14 0 top
C145  16.5,10 180 top
C146  27.39,11.97 0 top
C147  27.39,13.97 0 top
C148  32.22,7.02 180 top
C149  26.39,9.97 180 top
C150  22.41,12 0 top
C151  22.41,14 0 top
C152  21.41,10 180 top
C160  82.55,46.98 90 top
C161  78.55,42.34 180 top
C162  76.69,51.25 0 top
C163  44.66,22.17 270 bottom
C164  53.66,34.67 90 bottom
C165  54.66,32.17 180 bottom
C166  44.66,34.67 90 bottom
C167  43.66,32.17 0 bottom
C168  53.66,22.17 270 bottom
C169  54.66,24.67 180 bottom
C170  43.66,24.67 0 bottom
C200  4.65,13.53 180 top
C201  13.28,20.98 180 top
C202  10,45 180 top
C203  10,43 0 top
C204  12.2,33.04 90 bottom
C205  15.46,30.39 180 top
C206  15.41,31.67 180 top
C207  18.43,33.1 135 bottom
C208  22.37,37 315 bottom
C209  21.62,34.14 225 top
C210  19.14,36.11 225 top
C211  15.63,26.6 0 top
C301  68.29,30.51 270 top
D1  12.5,44 90 top
F200  8.5,15.75 180 top
F201  4,15.75 180 top
F202  8.5,40 180 top
F203  4,40 180 top
IC100  76.55,19.62 90 top
IC101  76.55,5.93 90 top
IC102  76.55,32.87 90 top
IC103  76.55,46.56 90 top
IC200  27,29 180 top
IC300  34.39,11.84 90 top
IC301  65.57,30.25 180 top
IC400  49.16,28.28 180 top
JP1  32.57,52.61 0 top
JP2  45,3 180 top
L1  5,25.5 180 bottom
L140  13,7 90 top
L141  18,7 90 top
L142  27.89,6.97 90 top
L143  22.91,7 90 top
LED1V2  70.55,45.87 180 top
LED2V5  70.55,32.87 180 top
LED3V3A  70.55,5.87 180 top
LED3V3B  70.55,18.87 180 top
LED801  66,53 0 top
LED802  68,53 0 top
LED803  66,3 180 top
LED804  68,3 180 top
R100  73.55,42.17 0 top
R101  70.59,10.74 90 top
R102  70.69,23.49 90 top
R103  70.55,37.87 90 top
R104  70.55,50.87 90 top
R201  15.75,28.04 180 top
R202  4,28 90 bottom
R203  6,28 90 bottom
R301  13.95,49.19 0 bottom
R302  10.45,49.15 0 bottom
R404  26.19,47.54 270 bottom
R405  67.67,23.4 270 top
R800  66,49 270 top
R801  68,49 270 top
R802  66,8 90 top
R803  68,8 90 top
T201  6,21 270 top
T202  6,34 270 top
X201  4.4,9 180 top
X202  4.4,46 180 top

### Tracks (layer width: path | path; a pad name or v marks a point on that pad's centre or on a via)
3V3A
  Top 0.254: IC301.1 IC301.4
  Top 0.406: C301.2 67.23,29.66 IC301.1
+1V2  (via drill 0.6)
  Top 0.254: IC400.73 41.2,37.03 | 41.2,37.03 41.3,37.03 | IC400.70 41.41,37.13 41.3,37.03 | 41.22,37.02 41.2,37.03 | IC400.78 v41.49,34.53 | v41.49,34.53 | IC400.84 41.46,31.53 v41.46,31.5 | IC400.102 v41.54,22.53 v41.55,22.52 41.55,21.27 40.41,20.12 IC400.109 | IC400.116 43.91,20.05 v43.92,20.06 | IC400.124 47.91,20.17 v47.94,20.2 | IC400.134 52.91,20.12 v52.93,20.14 | IC400.138 54.91,20.13 v54.89,20.14 54.96,20.2 56.57,20.2 57.24,19.53 IC400.1 | IC400.5 v56.78,21.53 v56.78,21.54 | IC400.45 53.91,37.06 v53.64,36.79 | IC400.34 57.55,36.03 v57.41,36.18 IC400.38 IC400.37 57.96,39.09 v57.96,41.96 | IC400.29 57.44,33.53 v56.72,33.52 | IC400.61 45.91,36.64 v45.92,36.62 | v41.49,34.53 41.49,36.84 41.3,37.03 | v63.7,43.34 63.71,43.32 70.46,43.32 71.24,42.57 71.24,41.04 71.53,40.74 74.05,40.74 74.5,41.19 R100.2
  Top 0.406: R104.2 72.76,51.82 | 72.76,51.82 72.76,50.84 73.5,50.1 73.5,46.67 IC103.4 73.4,45.35 74.66,44.09 74.66,42.33 R100.2 77.53,42.17 C161.2 | 72.76,51.82 73.33,51.82 73.85,51.3 75.14,51.3 C162.+
  Bottom 0.254: 44.64,35.5 C166.2 | 43.43,21.3 44.65,21.3 C163.2 | 55.48,34.53 55.48,34.19 | 55.48,32.2 C165.2 | 53.7,21.36 C168.2 | C163.2 44.33,21.32 44.29,21.28 44.8,21.28 44.88,21.36 | 42.71,34.53 42.81,34.64 | 42.7,22.52 42.81,22.41 | v43.92,20.06 43.92,20.57 C163.2 | 47.94,21.29 47.91,21.32 | v52.93,20.14 52.93,20.58 C168.2 | v54.89,20.14 54.84,20.14 C168.2 | 53.64,35.54 C164.2 | v57.41,36.18 57.41,36.12 | v45.92,36.62 45.77,36.62
  Bottom 0.406: C167.2 C170.2 42.81,22.41 42.81,21.92 43.43,21.3 | C167.2 42.81,34.64 42.81,34.9 43.41,35.5 44.64,35.5 | 55.48,34.53 54.5,35.52 C164.2 C166.2 45.77,36.62 | 55.48,32.2 55.48,34.19 57.41,36.12 | 55.52,21.92 C169.2 C165.2 56.29,33.05 v56.72,33.52 | 55.52,21.92 54.95,21.36 53.7,21.36 | C168.2 47.91,21.32 C163.2 | v41.49,34.53 42.71,34.53 | v41.46,31.5 42.18,31.53 C167.2 | v41.55,22.52 42.7,22.52 | v47.94,20.2 47.94,21.29 | v56.78,21.54 55.9,21.54 55.52,21.92 | v53.64,36.79 53.64,35.54 | v63.7,43.34 59.34,43.34 v57.96,41.96
+2V5  (via drill 0.6)
  Top 0.254: IC400.107 v35.27,20.03 v35.26,20.04 | IC400.75 36.16,36.03 v35.28,36.76 | IC400.35 62.06,36.53 v62.1,36.55 | IC400.3 62.01,20.53 v62.02,20.51
  Top 0.406: IC102.4 73.4,32.38 | 73.4,32.38 73.4,31.7 | 73.4,31.7 73.4,29.53 74.5,28.42 75.65,28.42 C111.2 | R103.2 74.85,38.82 75.19,38.48 75.19,37.59 C112.+ 73.64,37.55 73.26,37.16 73.26,32.51 73.4,32.38 | v71.81,27.91 71.81,30.11 73.4,31.7
  Bottom 0.254: 34.05,20.14 C113.2 34.14,20.04 v35.26,20.04 | 63.41,36.92 63.31,36.83 63.31,36.7 | 63.31,36.7 63.57,36.44 | 63.21,36.55 C115.2 | 63.17,20.53 C114.2 | 63.35,18.22 63.31,18.25 | 63.31,36.7 C115.2 | C115.2
  Bottom 0.406: C113.2 C116.2 34.02,36.28 34.5,36.76 v35.28,36.76 | 34.05,20.14 34.05,18.03 37.52,14.57 42.15,14.57 43.7,13.03 60.48,13.03 62.03,14.57 63.31,15.88 63.31,18.25 C114.2 63.31,22.76 | C115.2 63.31,22.76 | v62.1,36.55 63.21,36.55 | v62.02,20.51 63.17,20.53 | v71.81,27.91 71.81,23.47 71.1,22.76 63.31,22.76
+3V3  (via drill 0.6)
  Top 0.406: v14.49,46.68 | v14.49,46.68 12.13,49.04 9.69,49.04 8.44,50.28 JP1.1
  Bottom 0.406: R203.2 6,29.86 7.48,31.34 7.48,36.89 8.64,38.05 8.64,39.14 10.58,41.07 10.58,46.62 9.5,47.7 R302.2 8.44,50.21 JP1.1 | R301.2 13,48.17 v14.49,46.68
+3V3A  (via drill 0.6)
  Top 0.254: IC400.81 38.32,33.03 38.27,33.09 v41.12,33.09 | IC400.93 41.09,27.03 v41.1,27.01 | IC400.117 44.41,19.06 v45.39,20.04 46.91,18.52 IC400.122 | IC400.130 50.91,19.56 v50.15,20.32 | IC400.139 55.41,15.84 v55.42,15.83 | IC400.17 57.88,27.53 v57.87,27.54 | IC400.26 57.81,32.03 v57.8,32.05 | IC400.62 45.41,38.29 44.63,37.52 v44.63,36.94 | IC400.56 48.41,37.08 v48.15,36.83 | IC400.47 52.91,37.66 v52.09,36.85 | IC400.40 56.41,37.25 v55.83,36.67 | 67.67,18.23 70.72,15.17 62.34,15.17 v61.14,16.37 | IC103.3 81.31,48.86 | v69.34,12.83 69.45,12.83 | v33.98,38.91 37.64,38.91 v37.86,39.13
  Top 0.406: C121.2 75.7,4.75 74.67,5.78 73.56,5.78 IC101.4 73.4,7.28 75.03,8.92 75.03,10.42 C122.+ 74.9,10.58 73.24,10.58 72.13,11.69 R101.2 | R405.2 67.67,18.23 70.61,15.29 70.61,11.7 R101.2 | C160.2 82.55,48.46 82.19,48.83 79.73,48.83 IC103.3 | 81.31,48.86 v82.39,49.95 | 69.45,12.83 R101.2
  Bottom 0.254: 56.74,39.24 C129.2 | C123.2 37.6,33.09 | C134.2 37.86,27.01 | C130.2 C132.2 48.7,17.52 48.68,17.53 | 50.15,17.55 50.12,17.52 | v57.87,27.54 59.45,27.54 C124.2 | 44.63,39.28 C133.2 | 48.15,39.3 C125.2 | 60.31,18.19 60.16,18.04 | 56.81,17.55 56.69,17.68 | 56.69,17.68 | 56.69,17.68 56.46,17.45
  Bottom 0.305: v61.14,16.37 61.14,17.06 60.16,18.04
  Bottom 0.406: C128.2 C124.2 60.31,18.19 | C128.2 60.31,38.07 59.14,39.24 56.74,39.24 | C127.2 C129.2 55.83,38.48 v55.83,36.67 | C127.2 C125.2 C133.2 39.33,39.32 38.65,38.63 | 38.65,38.63 37.51,37.49 C123.2 C134.2 37.51,19.29 39.27,17.53 48.68,17.53 | 48.7,17.52 50.12,17.52 C126.2 C131.2 55.42,16.27 v55.42,15.83 | v41.12,33.09 37.6,33.09 | v41.1,27.01 37.86,27.01 | v45.39,20.04 45.39,18.24 C130.2 | v50.15,20.32 50.15,17.55 | v57.8,32.05 59.19,32.05 C128.2 | v44.63,36.94 44.63,39.28 | v48.15,36.83 48.15,39.3 | v52.09,36.85 52.09,38.24 C127.2 | R404.2 26.19,44.87 26.45,44.61 28.28,44.61 v33.98,38.91 | 60.16,18.04 59.67,17.55 56.81,17.55 | v82.39,49.95 82.39,18.5 75.74,11.85 70.31,11.85 v69.34,12.83 | v37.86,39.13 38.15,39.13 38.65,38.63
+3V3B  (via drill 0.6)
  Top 0.254: v73.61,15.15 73.61,19.41 IC100.4
  Top 0.305: 31.23,0.65 57.3,0.64 v58.59,1.78
  Top 0.406: L140.1 L141.1 L143.1 27.86,5.9 L142.1 27.89,3.98 31.23,0.65 | C101.2 73.83,14.93 v73.61,15.15 | v59.48,9.93 59.48,6.61 58.65,5.78 58.65,1.83 v58.59,1.78 | R102.2 72.61,24.44 73.04,24.02 75.19,24.02 C102.+ 75.19,20.21 74.6,19.62 IC100.4
  Bottom 0.254: 73.56,15.1 v73.61,15.15 | 65.73,9.95 65.72,9.95
  Bottom 0.406: 65.72,9.95 v59.48,9.93 | 73.56,15.1 70.31,15.1 68.29,13.25 68.29,10.31 67.94,9.95 65.73,9.95
+5V  (via drill 0.6)
  Top 0.406: 9.77,53.88 9.75,53.91 9.75,55.27 83.75,55.22 84.07,54.9 84.07,35.7 84.15,35.7 84.15,33.96 | C120.2 82.55,7.69 | 82.55,7.69 81.97,8.27 79.73,8.27 IC101.3 79.6,8.33 79.6,9.05 80.06,9.52 v81.79,9.52 84.09,9.52 84.09,9.51 | 84.2,9.34 84.15,9.29 | 84.15,9.29 82.55,7.69 | C100.2 82.55,34.87 | 82.55,34.87 82.07,35.35 79.88,35.35 IC102.3 | 84.15,33.96 84.15,21.68 | 84.15,21.68 84.15,9.29 | 82.55,34.87 82.59,34.87 82.59,33.96 84.15,33.96 | IC100.3 81.05,21.92 81.4,21.57 82.54,21.57 C110.2 84.04,21.57 84.15,21.68
  Top 0.813: JP1.4 9.77,53.88 JP1.2 | JP2.2 JP2.1
  Bottom 0.406: R202.2 4.29,29.25 4.29,29.71 6,31.42 6,38.91 7.57,40.48 8.73,40.48 9.79,41.54 9.79,45.89 9.7,45.98 7.02,45.98 4.43,48.57 4.43,50.09 5.8,51.22 5.8,52.81 7.3,53.88 JP1.2 | JP2.1 56.43,6.83 57.65,8.05 80.33,8.05 v81.79,9.52
AVDD_ADC  (via drill 0.6)
  Top 0.254: IC200.40 22.59,29.23 17.94,29.23 v17.8,29.38 | v19.88,31.76 22.59,31.76 IC200.35
  Top 0.406: L140.2 13,8.61 12.57,9.05 12.57,9.93 C142.+ 12.5,10.55 12.89,10.94 12.89,11.96 C140.2 C141.2 12.85,16.25 13.57,16.97 16.32,16.97 v16.61,17.27
  Bottom 0.406: v16.61,17.27 16.61,27.73 16.62,28.45 16.86,28.45 v17.8,29.38 17.8,29.68 v19.88,31.76
AVDD_DAC  (via drill 0.6)
  Top 0.254: IC200.43 20.86,27.75 v20.38,27.27
  Top 0.406: v17.85,15.25 C144.2 C143.2 17.85,10.15 C145.+ L141.2
  Bottom 0.406: v20.38,27.27 20.38,27 17.86,24.48 17.86,15.13 v17.85,15.25
CLK
  Top 0.254: IC200.57 27.25,21.56 27.25,20.75 27.25,19.81 28.25,18.8 29.83,18.8 32.28,16.36 IC300.4
CLKVDD  (via drill 0.6)
  Top 0.254: v28.08,21.5 28.08,21.57 27.74,21.92 27.74,24.6 IC200.58
  Top 0.406: v27.77,16.01 28.24,15.54 C147.2 C146.2 28.24,10.97 27.89,10.62 C149.+ L142.2 29.8,8.07 29.88,7.99 | IC300.6 30.58,9.3 29.88,8.6 29.88,7.99 | 29.88,7.99 29.88,7.63 30.42,7.09 31.3,7.09 C148.2
  Bottom 0.406: v27.77,16.01 27.77,21.19 v28.08,21.5
DEBUG_1  (via drill 0.6)
  Top 0.254: IC400.30 64.63,34.03 65.95,35.35 65.95,35.39 68.49,37.93 68.49,41.51 v69.27,42.28 | 65.95,48.01 R800.2 65.98,48.03
  Top 0.406: v65.98,46 65.98,48.03
  Bottom 0.406: v69.27,42.28 69.27,42.72 v65.98,46
DEBUG_2  (via drill 0.6)
  Top 0.254: IC400.28 66.48,33.03 69.13,35.68 69.13,40.47 70.28,41.62 v70.31,41.62 | 68.11,47.94 R801.2 | 68.11,45.5 v68.17,45.44
  Top 0.406: 68.11,47.94 68.11,45.5
  Bottom 0.254: 70.28,41.64 v70.31,41.62
  Bottom 0.406: v68.17,45.44 68.17,44.72 70.28,42.61 70.28,41.64
DEBUG_3  (via drill 0.6)
  Top 0.254: IC400.4 61.21,21.03 61.35,21.18 61.35,21.19 61.47,21.3 62.54,21.3 66.03,17.81 v66.03,16.12 | v66,13.72 v66,13.73
  Top 0.406: R802.2 v66,13.72
  Bottom 0.254: 66,16.09 v66.03,16.12
  Bottom 0.406: v66,13.73 66,16.09
DEBUG_4  (via drill 0.6)
  Top 0.254: IC400.6 62.55,22.03 67.77,16.81 v68,16.58 | 68,14.26 v68.01,14.27
  Top 0.406: R803.2 68,14.26
  Bottom 0.254: 68.01,16.57 v68,16.58
  Bottom 0.406: v68.01,14.27 68.01,16.57
DVDD  (via drill 0.6)
  Top 0.254: IC200.60 28.75,22.65 v28.73,22.64 | IC200.64 30.75,23.16 | 30.75,23.16 30.75,22.65 v30.73,22.64 30.73,23.14 30.75,23.16 | IC200.17 30.75,34.84 v31.05,35.09
  Top 0.406: v23.26,15.31 23.26,15.1 C151.2 C150.2 23.27,11.98 23.27,11.07 22.91,10.7 C152.+ L143.2
  Bottom 0.406: v28.73,22.64 29.92,22.64 | 29.92,22.64 v30.73,22.64 31.05,23.22 v31.05,35.09 | 29.92,22.64 29.81,22.52 29.81,15.86 29.07,15.12 23.45,15.12 v23.26,15.31
FPGA_ADIO00
  Top 0.254: IC200.12 33.76,30.75 35.04,32.03 IC400.83
FPGA_ADIO01
  Top 0.254: IC200.11 34.15,30.25 34.93,31.03 IC400.85
FPGA_ADIO02
  Top 0.254: IC400.86 35.19,30.53 34.41,29.75 IC200.10
FPGA_ADIO03
  Top 0.254: IC200.9 34.64,29.25 35.42,30.03 IC400.87
FPGA_ADIO04
  Top 0.254: IC400.98 37.6,24.55 34.12,28.75 IC200.8
FPGA_ADIO05
  Top 0.254: IC400.99 37.43,24.04 33.95,28.24 IC200.7
FPGA_ADIO06
  Top 0.254: IC400.100 37.23,23.54 33.77,27.74 IC200.6
FPGA_ADIO07
  Top 0.254: IC400.101 37.06,23.04 33.58,27.25 IC200.5
FPGA_ADIO08
  Top 0.254: IC400.103 37.19,22.04 33.42,26.74 IC200.4
FPGA_ADIO09
  Top 0.254: IC200.3 33.19,26.24 36.98,21.54 IC400.104
FPGA_ADIO10
  Top 0.254: IC200.2 32.97,25.75 36.71,21.03 IC400.105
FPGA_ADIO11
  Top 0.254: IC200.1 32.8,25.25 36.46,20.53 IC400.106
FPGA_CE0_SPI0
  Top 0.254: IC400.43 54.91,43.75 50.46,48.19 39.62,48.19 37.64,50.17
  Top 0.406: 37.64,50.17 37.64,52.63 JP1.24
FPGA_CE0_SPI1
  Top 0.254: IC400.50 51.41,43.47 48.52,46.35 25.51,46.35 22.43,49.43
  Top 0.406: 22.43,49.43 22.43,52.59 JP1.12
FPGA_CE1_SPI0
  Top 0.254: IC400.42 55.41,43.91 50.56,48.75 41.25,48.75 40.13,49.87
  Top 0.406: 40.13,49.87 40.13,52.67 JP1.26
FPGA_CE1_SPI1
  Top 0.254: IC400.51 50.91,43.25 48.03,45.93 24.22,45.93 21.09,49.06 | 21.09,51.29 JP1.11
  Top 0.406: 21.09,49.06 21.09,51.29
FPGA_CE2_SPI1
  Top 0.254: 54.68,48.43 55.55,48.43 63.96,40.02 63.96,36.56 62.94,35.53 IC400.33
  Top 0.406: JP1.36 51.82,53.88 52.88,52.82 52.88,50.23 54.68,48.43
FPGA_CLKOUT
  Top 0.254: IC400.72 40.41,40.29 39.77,40.92 32.83,40.92 29.75,37.84 IC200.19
FPGA_CLOCK
  Top 0.254: IC400.25 64.53,31.53 IC301.3
FPGA_CONF_DONE  (via drill 0.6)
  Top 0.254: IC400.92 36.87,27.53 v35.7,28.7
  Top 0.406: v24.64,48.87 25.4,48.87 26.13,49.6 26.13,51.25 JP1.15
  Bottom 0.254: v35.7,28.7 35.7,28.72 | 26.23,48.54 R404.1
  Bottom 0.305: 35.13,35.38 36.4,36.65 36.4,40.57 28.42,48.54
  Bottom 0.406: 35.7,28.72 34.76,29.71 34.76,34.23 35.13,34.93 35.13,35.38 | 28.42,48.54 26.23,48.54 24.97,48.54 v24.64,48.87
FPGA_DATA[0]  (via drill 0.6)
  Top 0.254: IC400.13 64.72,25.53 66.33,27.14 67.53,27.14 v67.61,27.22
  Bottom 0.254: JP1.33 49.23,51.34 51.83,48.74 61.3,48.74 67.61,42.43
  Bottom 0.406: 67.61,42.43 v67.61,27.22
FPGA_DCLK  (via drill 0.6)
  Top 0.254: v65.76,25.03 64.76,25.03 64.07,25.03 IC400.12
  Bottom 0.254: JP1.18 28.9,53.88 | 30.94,48.42 | 61.02,48.19 66.78,42.46 66.78,27.7 65.76,26.68
  Bottom 0.406: 28.9,53.88 29.97,52.81 29.97,49.39 30.94,48.42 | 30.94,48.42 31.17,48.19 61.02,48.19 | v65.76,25.03 65.76,26.68
FPGA_MISO_SPI0
  Top 0.254: IC400.46 53.41,43.59 49.66,47.34 35.74,47.34 33.79,49.29 | 33.79,51.29 JP1.21
  Top 0.406: 33.79,49.29 33.79,51.29
FPGA_MISO_SPI1
  Top 0.254: IC400.39 56.91,43.94 51.69,49.15 | 51.69,51.28 JP1.35
  Top 0.406: 51.69,49.15 51.69,51.28
FPGA_MODE  (via drill 0.6)
  Top 0.254: IC400.110 40.91,15.02 v38.75,12.85 | v19.17,12.09 19.17,15.17 21.13,17.13 22.54,17.13 25.25,19.84 IC200.53
  Bottom 0.254: v38.75,12.85 38.98,13.08
  Bottom 0.406: 38.98,13.08 37.67,11.77 19.43,11.77 v19.17,12.09
FPGA_MOSI_SPI0
  Top 0.254: IC400.49 51.91,43.8 48.84,46.87 33.46,46.87 31.36,48.97 | 31.36,51.29 JP1.19
  Top 0.406: 31.36,48.97 31.36,51.29
FPGA_MOSI_SPI1
  Top 0.254: IC400.32 63.5,35.03 64.47,36 64.47,40.4 58.15,46.72 58.15,52.18 57.87,52.68
  Top 0.406: JP1.38 54.16,53.62 55.33,52.68 57.87,52.68
FPGA_NCONFIG  (via drill 0.6)
  Top 0.254: v64.65,27.14 | v64.65,27.14 63.53,26.03 IC400.14
  Bottom 0.254: 60.87,47.47 66.26,42.08 66.26,28.76
  Bottom 0.406: JP1.13 24.61,51.34 24.93,51.01 24.93,50.17 25.32,49.78 28.7,49.78 31.02,47.47 60.87,47.47 | 66.26,28.76 v64.65,27.14
FPGA_NSTATUS  (via drill 0.6)
  Top 0.254: v67.88,25.8 67.88,25.74 67.84,25.05 67.84,24.52 R405.1 67.58,24.26 66.69,24.26 65.96,23.53 IC400.9
  Bottom 0.254: JP1.37 54.16,50.11 54.96,49.31 61.56,49.31 68.1,42.78 68.47,42.4 68.47,26.38 | v67.88,25.8 v67.89,25.8
  Bottom 0.406: v67.89,25.8 68.47,26.38
FPGA_PGA0
  Top 0.254: IC200.29 24.75,38.78 30.8,44.84 45.28,44.84 46.91,43.22 IC400.59
FPGA_PGA1
  Top 0.254: IC200.28 25.25,38.57 31.07,44.37 44.93,44.37 46.41,42.9 IC400.60
FPGA_PGA2
  Top 0.254: IC200.27 25.75,38.42 31.3,43.96 42.04,43.96 44.41,41.62 IC400.64
FPGA_PGA3
  Top 0.254: IC200.26 26.25,38.23 31.54,43.52 41.71,43.52 43.91,41.32 IC400.65
FPGA_PGA4
  Top 0.254: IC200.25 26.75,38.07 31.78,43.1 41.41,43.08 43.41,41.07 IC400.66
FPGA_PGA5
  Top 0.254: IC200.24 27.25,37.97 31.94,42.65 41.16,42.65 42.91,40.91 IC400.67
FPGA_RESET
  Top 0.254: IC200.30 24.25,38.99 30.62,45.36 45.7,45.36 47.41,43.66 IC400.58
FPGA_RXCLK
  Top 0.254: IC200.16 32.54,32.75 35.32,35.53 IC400.76
FPGA_RXEN
  Top 0.254: IC200.13 33.46,31.25 35.74,33.53 IC400.80
FPGA_SCLK
  Top 0.254: IC200.22 28.25,38.32 32.17,42.23 40.96,42.23 42.41,40.78 IC400.68
FPGA_SCLK_SPI0
  Top 0.254: IC400.44 54.41,43.47 50.11,47.77 37.88,47.77 36.38,49.26 | JP1.23
  Top 0.406: 36.38,49.26 JP1.23
FPGA_SCLK_SPI1
  Top 0.254: 58.7,53.29 58.7,47 65.21,40.49 65.21,35.63 64.11,34.53 IC400.31
  Top 0.406: JP1.40 58.1,53.88 58.7,53.29
FPGA_SDIO
  Top 0.254: IC200.20 29.25,37.99 32.63,41.37 39.96,41.37 40.91,40.43 IC400.71
FPGA_SDO
  Top 0.254: IC200.21 28.75,38.19 32.35,41.78 40.64,41.78 41.91,40.52 IC400.69
FPGA_TXCLK
  Top 0.254: IC200.15 32.98,32.25 35.76,35.03 IC400.77
FPGA_TXEN
  Top 0.254: IC200.14 33.21,31.75 35.49,34.03 IC400.79
GND  (via drill 0.6, 2)
  Top 0.254: IC400.95 IC400.94 39.28,26.53 40.23,25.58 44.02,25.58 46.69,28.25 47.41,28.25 | IC400.97 IC400.96 | IC400.108 36.72,19.53 36.38,19.19 36.38,14.48 IC300.3 36.49,15.78 33.92,18.35 32.19,18.35 | IC400.123 47.41,19.26 46.5,20.17 46.5,25.62 48.3,27.42 | 48.3,27.42 IC400.E | 47.41,28.25 47.44,28.28 | 48.3,27.42 48.24,27.42 47.41,28.25 | IC200.36 24.75,31.25 | 24.75,31.25 26.14,29.86 | 26.14,29.86 IC200.65 | IC200.39 26.03,29.75 26.14,29.86 | IC200.44 25.25,27.25 | 25.25,27.25 25.64,27.64 | 25.64,27.64 26.25,28.25 | 25.25,27.25 23.75,25.75 IC200.47 IC200.48 20.64,25.25 20.27,24.89 20.27,23.77 v20.35,23.7 v20.35,20.9 | IC200.54 25.75,27.54 25.64,27.64 | IC200.55 26.25,28.25 | 26.25,28.25 IC200.65 | 28.25,27.75 29.75,26.25 IC200.62 29.74,24.59 29.74,23.73 29.83,23.64 29.83,20.71 32.19,18.35 | IC200.59 28.25,27.75 | 28.25,27.75 IC200.65 | IC200.31 23.75,32.25 24.75,31.25 | 24.75,31.25 24.75,31.69 24.81,31.76 24.32,32.25 IC200.34 21.2,32.24 20.39,32.91 17.4,32.91 14.71,35.6 11.22,39.1 8.55,39.1 F202.2@2 | IC200.63 30.25,25.71 26.92,29.04 26.92,29.07 30.25,32.41 IC200.18 30.26,33.41 30.26,36.12 32.02,37.54 35.98,37.55 36.55,36.53 IC400.74 39.76,36.53 v40.2,36.09 | 67.43,31.5 67.6,31.33 | 68.25,31.33 C301.1 | LED2V5.C | C141.1 11.15,14.04 11.22,14.11 | IC400.131 51.41,15.8 v50.53,15.82 | IC400.E 51.02,26.42 51.02,25.56 55.9,20.68 57.48,20.68 58.13,20.03 IC400.2 61.13,20.03 61.84,19.32 | IC400.140 55.91,18.47 56.26,18.82 58.26,18.82 58.93,18.15 61.33,18.15 | IC400.36 60.81,37.03 61.28,37.5 61.28,40.3 v60.87,40.71 | IC400.82 39.98,32.53 40.2,32.3 47.86,32.3 49.22,30.95 49.22,29.32 | 49.22,29.32 49.22,28.34 IC400.E
  Top 0.254: IC400.21 50.55,29.53 | 50.55,29.53 50.39,29.53 | 50.39,29.53 v49.19,28.33 | IC400.19 49.41,28.53 IC400.E | IC301.2 66.54,31.52 66.54,32.2 66.21,32.53 IC400.27 58.75,32.53 58.41,32.88 57.28,32.88 56.94,32.54 54.46,32.54 54.01,32.99 | v68.99,18.68 68.99,18.21 69.45,17.75 70.48,17.75 LED3V3B.C | IC400.57 47.91,41.17 v49.24,42.5 | 50.39,29.53 50.78,29.92 50.78,36.96 51.62,37.8 52.21,37.8 52.41,37.99 IC400.48 | IC400.41 55.91,37.97 55.61,37.67 55.41,37.67 54.67,36.94 54.67,33.65 54.01,32.99 | 54.01,32.99 50.55,29.53 | IC400.63 44.91,38.39 44.68,38.16 44.22,38.16 43.46,37.4 43.46,36.47 | 43.46,36.47 43.46,36.06 45.7,33.82 48.58,33.82 49.26,33.14 49.26,29.36 49.22,29.32 | 61.84,19.32 61.84,18.66 61.33,18.15 | 61.84,19.32 62.22,19.32 62.9,18.65 63.6,18.65 v64.9,17.35 | 72.62,42.19 R100.1 | IC400.118 44.91,14.17 v44.48,13.91 | 61.33,18.15 61.33,18.03 v61.88,17.48 | 32.19,18.35 32.19,17.93 v32.51,17.61 | v25.11,2.36 19.83,2.36 14.43,2.36 12.3,2.36 8.27,6.38 | v5.89,17.65 5.89,18.57 5.73,18.74 | v9.82,25.21 9.82,26.45 9.98,26.6 | v9.78,28.62 9.78,26.66 9.71,26.6 | v42.6,36.6 43.33,36.6 43.46,36.47
  Top 0.305: 15.52,36.06 15.52,36.07 | 14.71,35.6 15.17,36.06 15.51,36.06 v17.29,37.84 | v20.32,2.44 19.91,2.44 19.83,2.36 | 30.25,32.41 30.25,32.01 v29.19,30.95 | 26.14,29.86 26.14,30.02 v25.54,30.62 | 28.25,27.75 28.25,27.74 v28.32,27.67 | 25.25,27.25 25.25,27.34 v25.34,27.43 | v15.13,2.44 14.51,2.44 14.43,2.36 | 49.41,28.53 49.39,28.53 v49.19,28.33
  Top 0.406: IC400.96 IC400.95 | F200.2@2 F200.2@1 | R201.2 14.8,26.62 C211.1 9.98,26.6 9.71,26.6 9.09,26.6 7.64,25.15 7.64,23.41 | 7.64,23.41 7.64,22.88 8.28,22.24 13.81,22.24 14.18,21.86 14.18,21.04 C201.1 14.13,19.99 13.92,19.78 7.99,19.78 7.29,19.08 7.29,18.63 | 7.29,18.63 7.29,17 7.61,16.68 8.42,16.68 F200.2@1 | 7.29,18.63 7.19,18.74 5.73,18.74 5.13,18.74 4,17.61 F201.2@1 F201.2@2 3.81,14.71 2.42,14.71 1.85,14.13 X201.4 X201.3 X201.2 7.02,6.38 8.27,6.38 8.91,7.02 14.55,7.02 15.01,7.48 | T201.1 7.51,23.54 7.64,23.41 | X201.5 6.95,10.33 7.35,9.93 9.43,9.93 C142.- 9.55,10.05 9.55,11.45 10.1,12 C140.1 C141.1 | 4.05,43.45 X202.3 X202.4 X202.5 8.74,46.76 12.42,46.76 12.5,46.68 D1.B | 4.05,43.45 X202.2 6.95,41.38 7.41,40.92 8.43,40.92 F202.2@1 F202.2@2 | 4.05,43.45 4,43.4 F203.2@1 F203.2@2 4,38.27 4.62,37.66 4.62,33.1 3.01,31.5 2.23,31.5 T202.3 | LED801.C LED802.C | C147.1 C146.1 25.33,11.97 25.07,11.71 25.07,10.15 | 25.07,10.15 C149.- | C151.1 C150.1 20.26,12 19.91,11.64 C152.- | C152.- | C144.1 C143.1 16.15,10.26 15.9,10.01 C145.- | C145.- | IC301.2 67.43,31.5 | 67.6,31.33 68.25,31.33 | C301.1 69.07,31.36 69.52,31.82 LED2V5.C | LED803.C LED804.C 69.18,1.95 70.36,3.13 | 70.36,3.13 70.55,3.31 LED3V3A.C | 11.22,14.11 11.22,16.36 10.77,16.8 9.27,16.8 9.04,16.58 8.52,16.58 F200.2@1 | C145.- 15.01,7.48 | C152.- 19.91,7.21 | 19.91,7.21 19.72,7.02 15.46,7.02 15.01,7.48 | 25.07,10.15 25.07,7.34 | 25.07,7.34 24.78,7.05 20.07,7.05 19.91,7.21 | 25.07,7.34 25.93,7.34 26.26,7.02 28.92,7.02 31.71,4.23 33.53,4.23 JP2.19 33.08,4.76 C148.1 | 77.73,3.48 77.4,3.14 C121.1 77.4,1.13 76.99,0.72 72.77,0.72 70.36,3.13
  Top 0.406: 77.73,3.48 77.9,3.65 79.68,3.65 IC101.1 82,3.63 82.52,4.16 82.52,5.12 C120.1 | C101.1 79.28,14.93 | 79.28,14.93 79.69,14.52 79.69,11.97 79.58,11.97 C122.- 78.05,9.57 76.64,8.16 76.64,4.73 77.73,3.64 77.73,3.48 | C110.1 82.55,18.12 81.81,17.39 79.76,17.39 IC100.1 | 79.28,14.93 79.49,14.93 79.95,15.4 79.95,17.06 IC100.1 | C100.1 82.55,31.43 81.75,30.63 79.77,30.63 IC102.1 | IC100.1 79.66,17.35 78.05,17.35 77.23,18.17 77.23,22.29 77.96,23.02 77.96,23.77 C102.- 78.08,24.13 78.08,26.79 77.36,27.51 C111.1 79.31,28.41 79.77,28.87 79.77,30.49 IC102.1 | IC103.1 79.7,42.64 C161.1 79.43,42.31 79.43,40.59 78.14,39.3 C112.- 78.12,37.52 78.12,36.61 77.42,35.91 77.42,30.91 77.77,30.57 IC102.1 | IC103.1 81.83,44.26 82.51,44.94 82.51,46.09 C160.1 | LED802.C 64.15,54.05 v64.08,53.99 | 68.05,54 69.29,52.76 69.29,45.36 69.83,44.82 LED1V2.C 71.34,44.82 72.62,43.54 72.62,42.19 | IC200.65 26.96,29 26.92,29.04 | IC103.1 79.64,44.32 78.09,44.32 77.29,45.12 77.29,49.45 78.19,50.34 C162.- 78.19,52.91 77.1,54 68.05,54 | 68.05,54 LED802.C
  Top 0.813: JP2.20 JP2.19
  Bottom 0.254: 44.52,33.67 C166.1 | 53.66,32.32 C165.1 | 44.52,23.17 C163.1 | 53.66,24.52 C169.1 | C132.1 C130.1 44.48,15.63 | 44.48,41.2 C133.1 | C129.1 C127.1 | 61.95,33.23 C128.1 | 61.95,26.73 C124.1 62.1,26.58 | 56.74,15.74 C131.1 56.66,15.78 | 44.88,15.82 44.69,16.01 | C123.1 35.81,32.78 | 36.26,27.11 C134.1 | 35.53,15.74 | v50.53,15.82 50.53,15.8 50.79,15.82 | 49.24,41.04 49.26,41.02 | 61.41,38.8 61.28,38.92 | 62.6,17.72 62.53,17.79 | 35.65,26.49 35.8,26.64 35.97,26.64 36.04,26.72 | 64.9,20.55 C114.1 | 40.17,41.24 40.21,41.2 | v17.29,37.84 17.17,37.84 | 32.51,18.7 32.54,18.73 | 19.56,44.86 v19.65,44.76 19.65,44.65 | 22.59,41.82 v22.71,41.7 | 16.82,41.82 v16.8,41.8 | 16.8,39.78 16.77,39.74
  Bottom 0.305: 36.87,36.19 36.87,40.49 37.62,41.24 | 60.12,40.31 61.28,39.15 61.28,38.92 61.28,34.66 61.95,33.99 61.95,33.23 | 56.74,15.74 59.99,15.74 60.6,15.13 61.45,15.13 62.6,16.29 62.6,17.72 | 62.1,26.58 62.1,25.3 61.03,24.22 61.03,19.29 62.53,17.79 62.22,17.48 v61.88,17.48
  Bottom 0.406: 44.52,33.67 C167.1 C170.1 44.52,23.17 | C166.1 C164.1 53.66,32.32 | C163.1 C168.1 53.66,24.52 | C123.1 35.81,35.3 36.87,36.19 | 40.21,41.2 44.48,41.2 | C133.1 C125.1 49.26,41.02 C127.1 | C129.1 59.41,41.02 60.12,40.31 60.53,40.71 v60.87,40.71 | 61.95,33.23 61.95,26.73 | 56.66,15.78 56.03,14.75 53.92,14.75 C126.1 50.79,15.82 C132.1 44.88,15.82 | C116.1 C113.1 32.31,18.96 32.54,18.73 35.53,15.74 | 35.81,32.78 36.84,31.76 36.84,28.07 36.26,27.49 36.26,27.11 | JP1.6 13.52,52.95 | 13.52,52.95 13.31,52.73 13.14,52.73 13.01,52.6 7.55,52.6 6.6,51.54 6.6,49.35 X202.5 | 13.52,52.95 13.52,52.67 17.27,52.67 JP1.9 19.81,52.55 22.35,52.55 JP1.14 24.95,55.15 30.04,55.15 JP1.20 31.48,53.88 32.75,55.15 37,55.15 37.61,54.53 | 37.61,54.53 37.61,53.44 38.89,52.16 38.89,51.38 JP1.25 | 37.61,54.53 38.23,55.16 43.28,55.16 44,54.44 JP1.30 44.05,53.88 45.36,55.19 47.77,55.19 JP1.34 49.08,53.98 50.27,55.16 52.38,55.16 52.9,54.65 52.9,53.46 53.76,52.59 54.66,52.59 55.91,51.34 JP1.39 58.13,51.34 58.74,51.95 58.74,53.4 59.7,54.64 62.34,54.64 63.16,53.99 v64.08,53.99 | 35.53,15.74 37.42,13.85 40.04,13.85 40.36,13.53 40.36,13.15 | 40.36,13.15 40.36,11.96 36.38,7.99 35.05,7.99 33.66,6.59 33.66,5.06 33.22,4.62 JP2.19 | C207.1 17.82,32.66 14.81,35.67 14.81,37.79 16.02,38.99 | 16.02,38.99 16.77,39.74 20.82,39.74 C208.1 | 40.39,13.12 40.36,13.15 | C114.1 67,20.67 v68.99,18.68 | v49.24,42.5 49.24,41.04 | C115.1 65.02,37.88 64.1,38.8 61.41,38.8 | 44.69,16.01 38.19,16.01 36.38,17.82 36.38,24.86 35.65,25.6 35.65,26.49 | v64.9,17.35 64.9,20.55 | 37.62,41.24 40.17,41.24 | v44.48,13.91 44.48,15.63 | 17.17,37.84 16.02,38.99
  Bottom 0.406: v32.51,17.61 32.51,18.7 | C204.1 12.2,16.8 X201.5 | C165.1 53.81,30.1 52.25,28.53 49.39,28.53 v49.19,28.33 | v19.56,47.52 19.56,44.86 | 19.65,44.65 v16.8,41.8 16.8,39.78 | 22.59,41.82 v19.78,41.82 16.82,41.82 | v40.2,36.09 42.09,36.09 v42.6,36.6
  pour Top (isolate 0.61): 85.29,55.92 85.29,55.6 85.25,55.6 85.25,0.12 0.12,0.12 0.12,55.71
  pour Bottom (isolate 0.61): 85,55.71 85,55.7 84.91,55.7 84.91,0.39 0.39,0.39 0.39,0.42 0.34,0.42 0.36,55.69 0.36,55.71
IO-01
  Top 0.254: IC400.144 57.91,11.14 53.89,7.12 JP2.3 | JP2.3
IO-02
  Top 0.254: IC400.143 57.41,11.44 52.58,6.61 52.58,3.04 JP2.4
IO-03
  Top 0.254: IC400.142 56.91,12.06 51.39,6.54 51.39,4.31 JP2.5
IO-04
  Top 0.254: IC400.141 56.41,12.59 50.01,6.19 50.01,3.07 JP2.6
IO-05
  Top 0.254: IC400.136 53.91,11.62 48.76,6.48 48.76,4.32 JP2.7
IO-06
  Top 0.254: IC400.135 53.41,12.05 47.45,6.09 47.45,3.09 JP2.8
IO-07
  Top 0.254: IC400.133 52.41,12.34 46.29,6.22 46.29,4.29 JP2.9
IO-08
  Top 0.254: IC400.132 51.91,12.64 45.01,5.74 45.01,2.99 JP2.10
IO-09
  Top 0.254: IC400.125 48.41,10.84 43.73,6.16 JP2.11 | JP2.11
IO-10
  Top 0.254: IC400.121 46.41,10.05 42.45,6.09 42.45,3.02 JP2.12
IO-11
  Top 0.254: JP2.13 41.19,5.79 45.91,10.5 IC400.120
IO-12
  Top 0.254: IC400.119 45.41,10.97 39.94,5.5 39.94,2.98 JP2.14
IO-13
  Top 0.254: JP2.15 38.65,5.28 43.09,9.72 43.28,9.91 43.41,10.04 IC400.115
IO-14
  Top 0.254: IC400.114 42.91,10.27 38.66,6.03 37.7,6.03 37.41,5.74 37.41,2.97 JP2.16
IO-15
  Top 0.254: JP2.17 36.11,5.99 36.63,6.51 38.48,6.51 42.41,10.44 IC400.113
IO-16
  Top 0.254: IC400.112 41.91,10.6 38.4,7.09 35.75,7.09 34.91,6.25 34.91,2.93 JP2.18
N$1
  Bottom 0.406: R202.1 R203.1 6,25.6 L1.2
N$2
  Top 0.406: F203.3 2.58,36.92 T202.1
N$3
  Top 0.406: T202.4 10.01,31.46 11.12,30.34 14.57,30.34 C205.2
N$4
  Top 0.406: C201.2 9.83,20.98 T201.5
  Bottom 0.406: T201.5 6.74,21 5.06,22.67 5.06,23.43 3.84,24.66 3.84,25.44 L1.1
N$5
  Top 0.406: C202.1 C203.2 11.46,43 11.8,42.66 12.43,42.66 D1.A
N$6
  Top 0.254: IC200.50 23.75,19.73 22.65,18.63 9.98,18.63 T201.4
N$7
  Top 0.254: IC200.46 18.98,26.25 16.32,23.59 9.86,23.59 T201.6
N$8
  Top 0.406: T202.6 11.58,36.54 13,35.12 14.56,33.56 C206.2
N$10
  Top 0.406: R102.1 70.69,20.06 LED3V3B.A
N$11
  Top 0.406: LED2V5.A R103.1
N$13
  Top 0.254: IC200.37 19.46,30.75 18.51,31.7 16.29,31.7 C206.1
N$14
  Bottom 0.406: T202.5 12.09,34 C204.2
N$15
  Top 0.254: IC200.38 16.46,30.25 C205.1
N$16
  Top 0.406: LED801.A R800.1
N$17
  Top 0.406: LED802.A R801.1
N$18
  Top 0.406: LED803.A R802.1
N$19
  Top 0.406: LED804.A R803.1
N$20
  Top 0.406: R101.1 70.59,6.96 LED3V3A.A
N$23
  Top 0.406: LED1V2.A R104.1
N$25
  Top 0.406: F202.3 F203.1
N$28
  Top 0.406: X202.1 7.31,46 8.24,45.07 9.08,45.07 C202.2
N$29
  Top 0.406: C203.1 9.15,42.1 9.94,41.32 9.94,40.01 F202.1
N$30  (via drill 0.6)
  Top 0.254: IC200.33 21.81,32.75 C209.2
  Top 0.406: C210.2 19.44,35.12 19.7,34.86 v19.93,34.63 C209.2
  Bottom 0.254: C207.2 19.03,33.73
  Bottom 0.406: 19.03,33.73 v19.93,34.63
N$32  (via drill 0.6)
  Top 0.254: IC200.32 23.25,34.12 23.16,34.21 22.76,34.21 C209.1 22.03,34.67 | 21.16,35.57 21.1,35.62
  Top 0.406: 21.1,35.62 21.1,36.13 C210.1 | 21.16,35.57 v20.98,35.43 21.74,34.67 22.03,34.67
  Bottom 0.254: C208.2 21.5,36.14
  Bottom 0.406: 21.5,36.14 v20.98,35.43
N$33
  Top 0.254: IC200.42 19.45,28.25 17.76,26.57 16.52,26.57 C211.2
N$34
  Top 0.254: IC200.41 18.88,28.75 18.19,28.07 16.73,28.07 R201.1
N$69
  Top 0.406: X201.1 4.4,12.03 3.78,12.65 3.78,13.51 C200.2
N$71
  Top 0.406: C200.1 9.49,13.53 9.99,14.03 9.99,15.68 F200.1
N$72
  Top 0.406: F200.3 F201.1
N$73
  Top 0.406: T201.3 2.19,17.22 2.6,16.81 2.6,15.78 F201.3
SCL  (via drill 0.6)
  Top 0.406: v33.57,16.4 33.99,16.4 34.49,15.89 34.49,14.8 IC300.8
  Bottom 0.406: JP1.5 14.71,51.34 14.85,51.2 14.85,49.24 R301.1 14.9,48.07 15.98,46.99 15.98,46.2 14.09,43.68 14.14,17.78 15.43,16.29 15.38,14 16.21,13.17 30.34,13.17 v33.57,16.4
SDA  (via drill 0.6)
  Top 0.406: v29.97,10.39 30.1,10.39 30.2,10.59 34.1,10.59 34.36,10.04 34.36,9.01 IC300.7
  Bottom 0.406: JP1.3 11.66,50.66 11.66,49.41 R302.1 11.4,47.16 11.99,46.58 11.99,44.87 13.34,43.53 13.34,16.84 14.55,15.62 14.55,11.03 15.16,10.43 29.94,10.43 v29.97,10.39
SI570_OE
  Top 0.254: IC400.111 41.41,13.33 39.98,11.9 36.55,11.9 IC300.2

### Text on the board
tPlace: RX | RadioBerry | V1.0 | 18-12-2015 | TX | WWW.PA3GSB.NL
